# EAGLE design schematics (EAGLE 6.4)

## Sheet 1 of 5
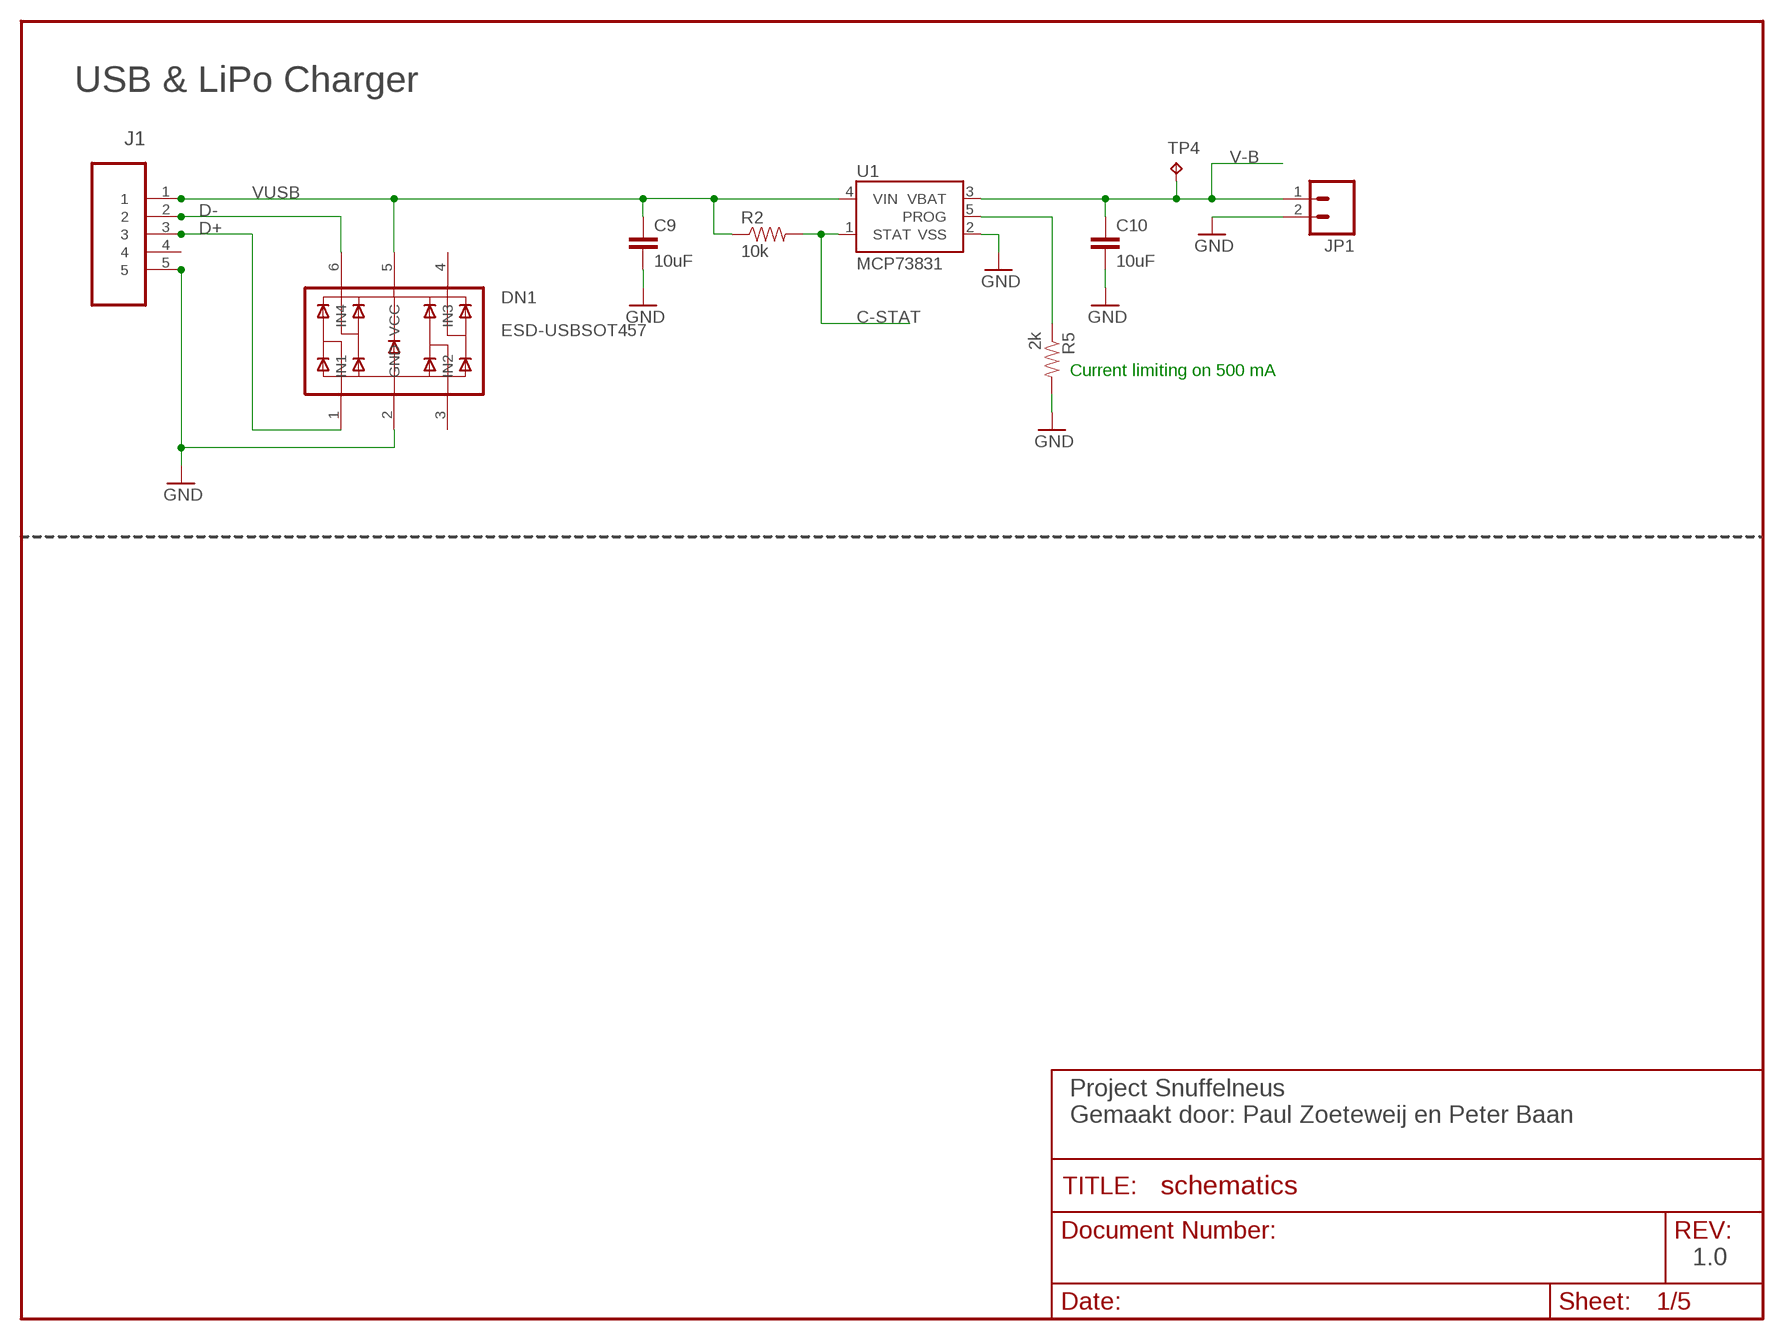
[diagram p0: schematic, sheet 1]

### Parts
C9  10uF  CAP0805  [0805]
C10  10uF  CAP0805  [0805]
DN1  ESD-USBSOT457  [SOT457]
J1  47346-0001  [MOLEX_47346-0001]
JP1  M02-JST-2MM-SMT  [S2B-PH]
R2  10k  RESISTOR  [0805]
R5  2k  RESISTOR  [0805]
TP4  TPTP20R  [TP20R]
U1  MCP73831  [SOT23-5]

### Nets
C-STAT: R2.2 U1.1(STAT) ; also sheet 3
D+: DN1.1(IN1) J1.3 ; also sheet 3
D-: DN1.6(IN4) J1.2 ; also sheet 3
GND: C9.2 C10.2 DN1.2(GND) J1.5 JP1.2 R5.2 U1.2(VSS) ; also sheet 2,3,4,5
N$11: R5.1 U1.5(PROG)
V-B: C10.1 JP1.1 TP4.TP U1.3(VBAT) ; also sheet 2
VUSB: C9.1 DN1.5(VCC) J1.1 R2.1 U1.4(VIN) ; also sheet 2
Unconnected: DN1.3(IN2) DN1.4(IN3) J1.4

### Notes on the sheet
- USB & LiPo Charger
- Current limiting on 500 mA
- Project Snuffelneus
  Gemaakt door: Paul Zoeteweij en Peter Baan
- 1.0

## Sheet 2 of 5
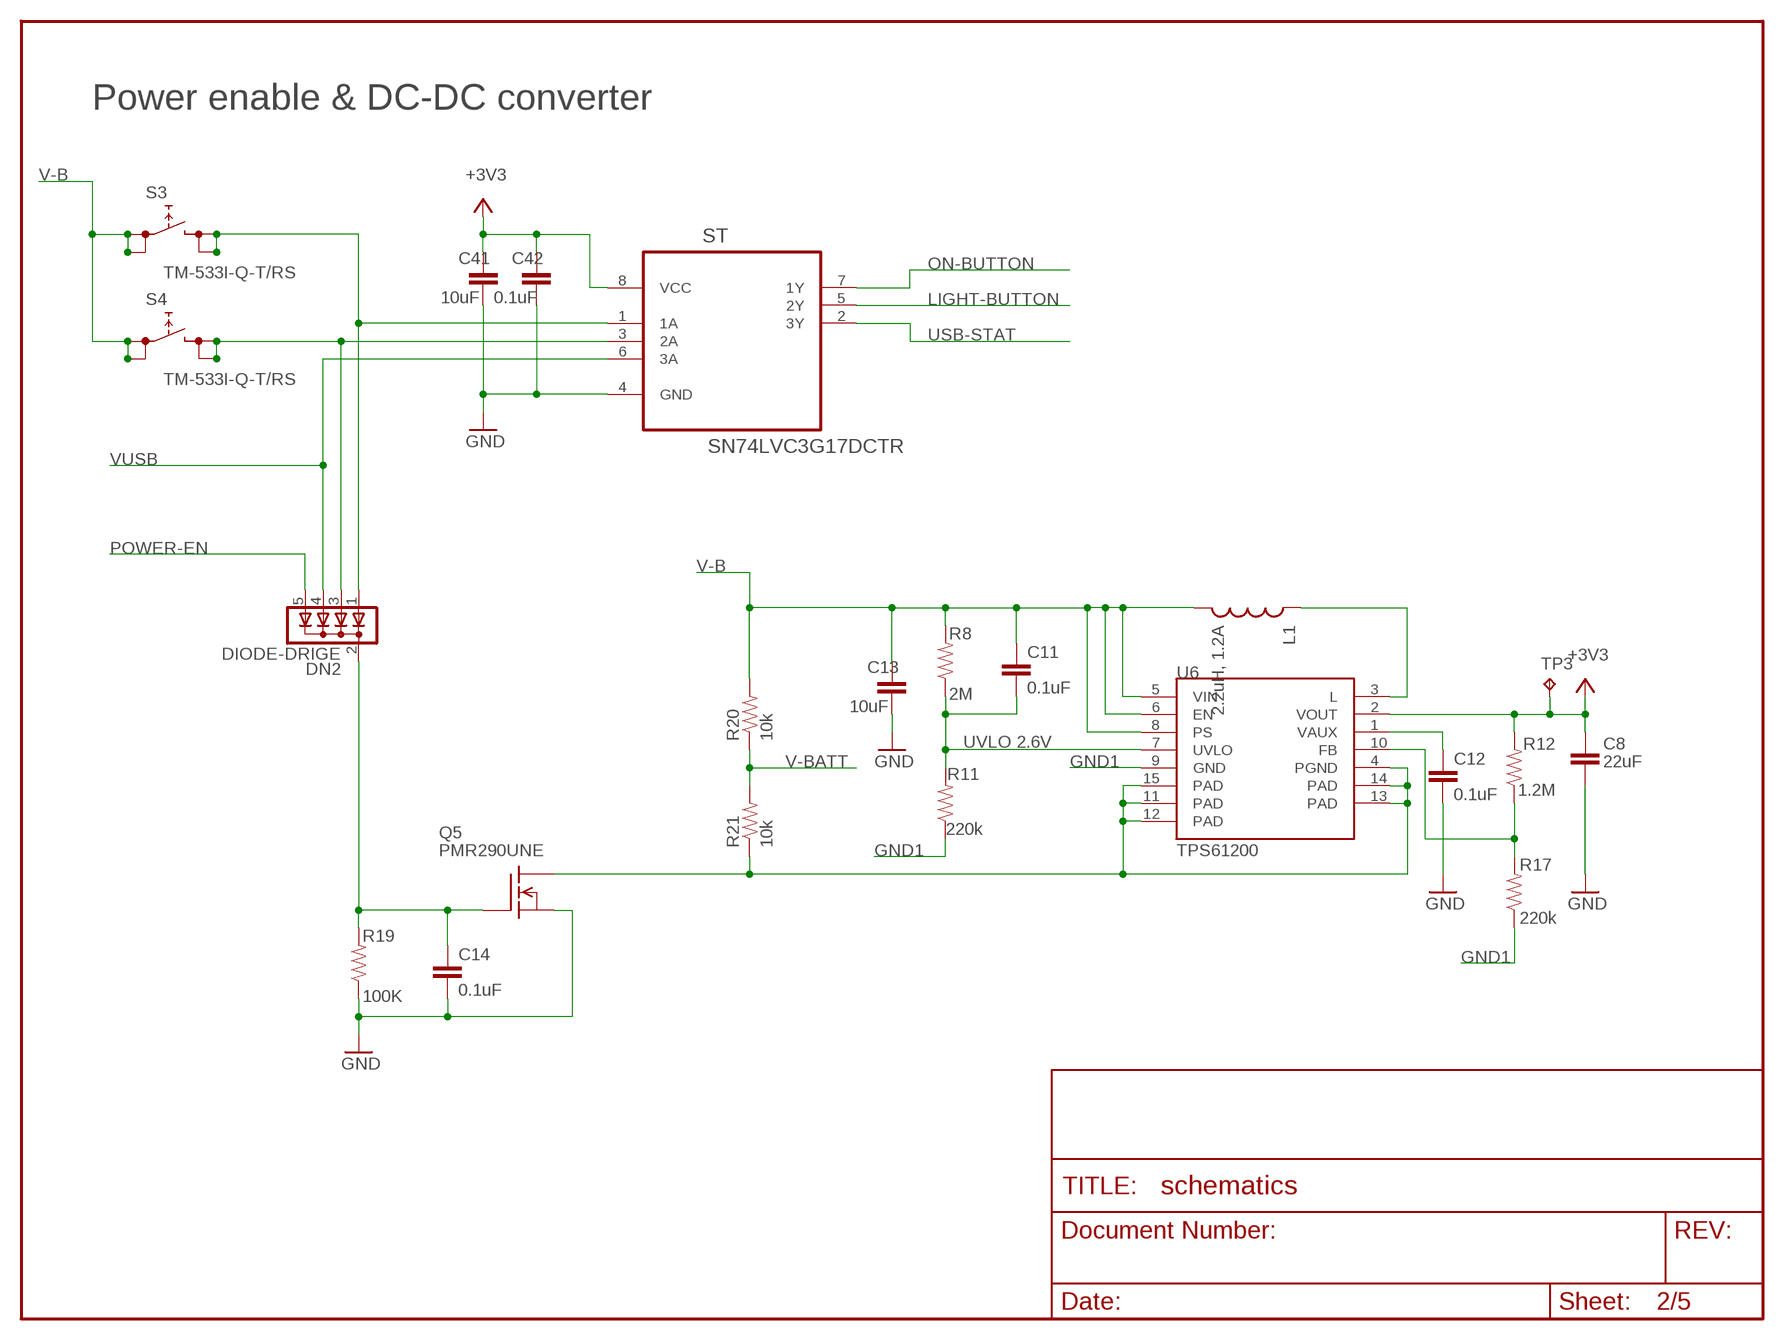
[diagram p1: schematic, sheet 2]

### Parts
C8  22uF  CAP0805  [0805]
C11  0.1uF  CAP0805  [0805]
C12  0.1uF  CAP0805  [0805]
C13  10uF  CAP0805  [0805]
C14  0.1uF  CAP0805  [0805]
C41  10uF  CAP0805  [0805]
C42  0.1uF  CAP0805  [0805]
DN2  DIODE-DRIGE  [SOT353]
L1  2.2uH, 1.2A  INDUCTORCR75  [LPS3015-222MLC]
Q5  PMR290UNE  [SOT23]
R8  2M  RESISTOR  [0805]
R11  220k  RESISTOR  [0805]
R12  1.2M  RESISTOR  [0805]
R17  220k  RESISTOR  [0805]
R19  100K  RESISTOR  [0805]
R20  10k  RESISTOR  [0805]
R21  10k  RESISTOR  [0805]
S3  TM-533I-Q-T/RS  [TM-533I-Q-T/R]
S4  TM-533I-Q-T/RS  [TM-533I-Q-T/R]
ST  SN74LVC3G17DCTR  [SOP65P400X130-8N]
TP3  TPTP20R  [TP20R]
U6  TPS61200  [QFN-10_PAD]

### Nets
3.3V1: R12.1 R17.2 U6.10(FB)
+3V3: C8.1 C41.1 C42.1 R12.2 ST.8(VCC) TP3.TP U6.2(VOUT) ; also sheet 3,4,5
GND: C8.2 C12.2 C13.2 C14.2 C41.2 C42.2 Q5.2(S) R19.1 ST.4(GND) ; also sheet 1,3,4,5
GND1: R11.1 R17.1 U6.9(GND)
LIGHT-BUTTON: ST.5(2Y) ; also sheet 3
LIGHT/WAKEUP-BUTTON1: DN2.3(A2) S4.T3 S4.T4 ST.3(2A)
N$8: L1.P$1 U6.3(L)
N$9: C12.1 U6.1(VAUX)
N$10: C14.1 DN2.2(C) Q5.1(G) R19.2
ON-BUTTON: ST.7(1Y) ; also sheet 3
PAD@4: Q5.3(D) R21.1 U6.4(PGND) U6.11(PAD) U6.12(PAD) U6.13(PAD) U6.14(PAD) U6.15(PAD)
POWER-EN: DN2.5(A4) ; also sheet 3
USB-STAT: ST.2(3Y) ; also sheet 3
UVLO1: C11.2 R8.1 R11.2 U6.7(UVLO)
V-B: C11.1 C13.1 L1.P$2 R8.2 R20.2 S3.T1 S3.T2 S4.T1 S4.T2 U6.5(VIN) U6.6(EN) U6.8(PS) ; also sheet 1
V-BATT: R20.1 R21.2 ; also sheet 3
VUSB: DN2.4(A3) ST.6(3A) ; also sheet 1
WAKEUP-BUTTON1: DN2.1(A1) S3.T3 S3.T4 ST.1(1A)

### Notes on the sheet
- Power enable & DC-DC converter
- UVLO 2.6V

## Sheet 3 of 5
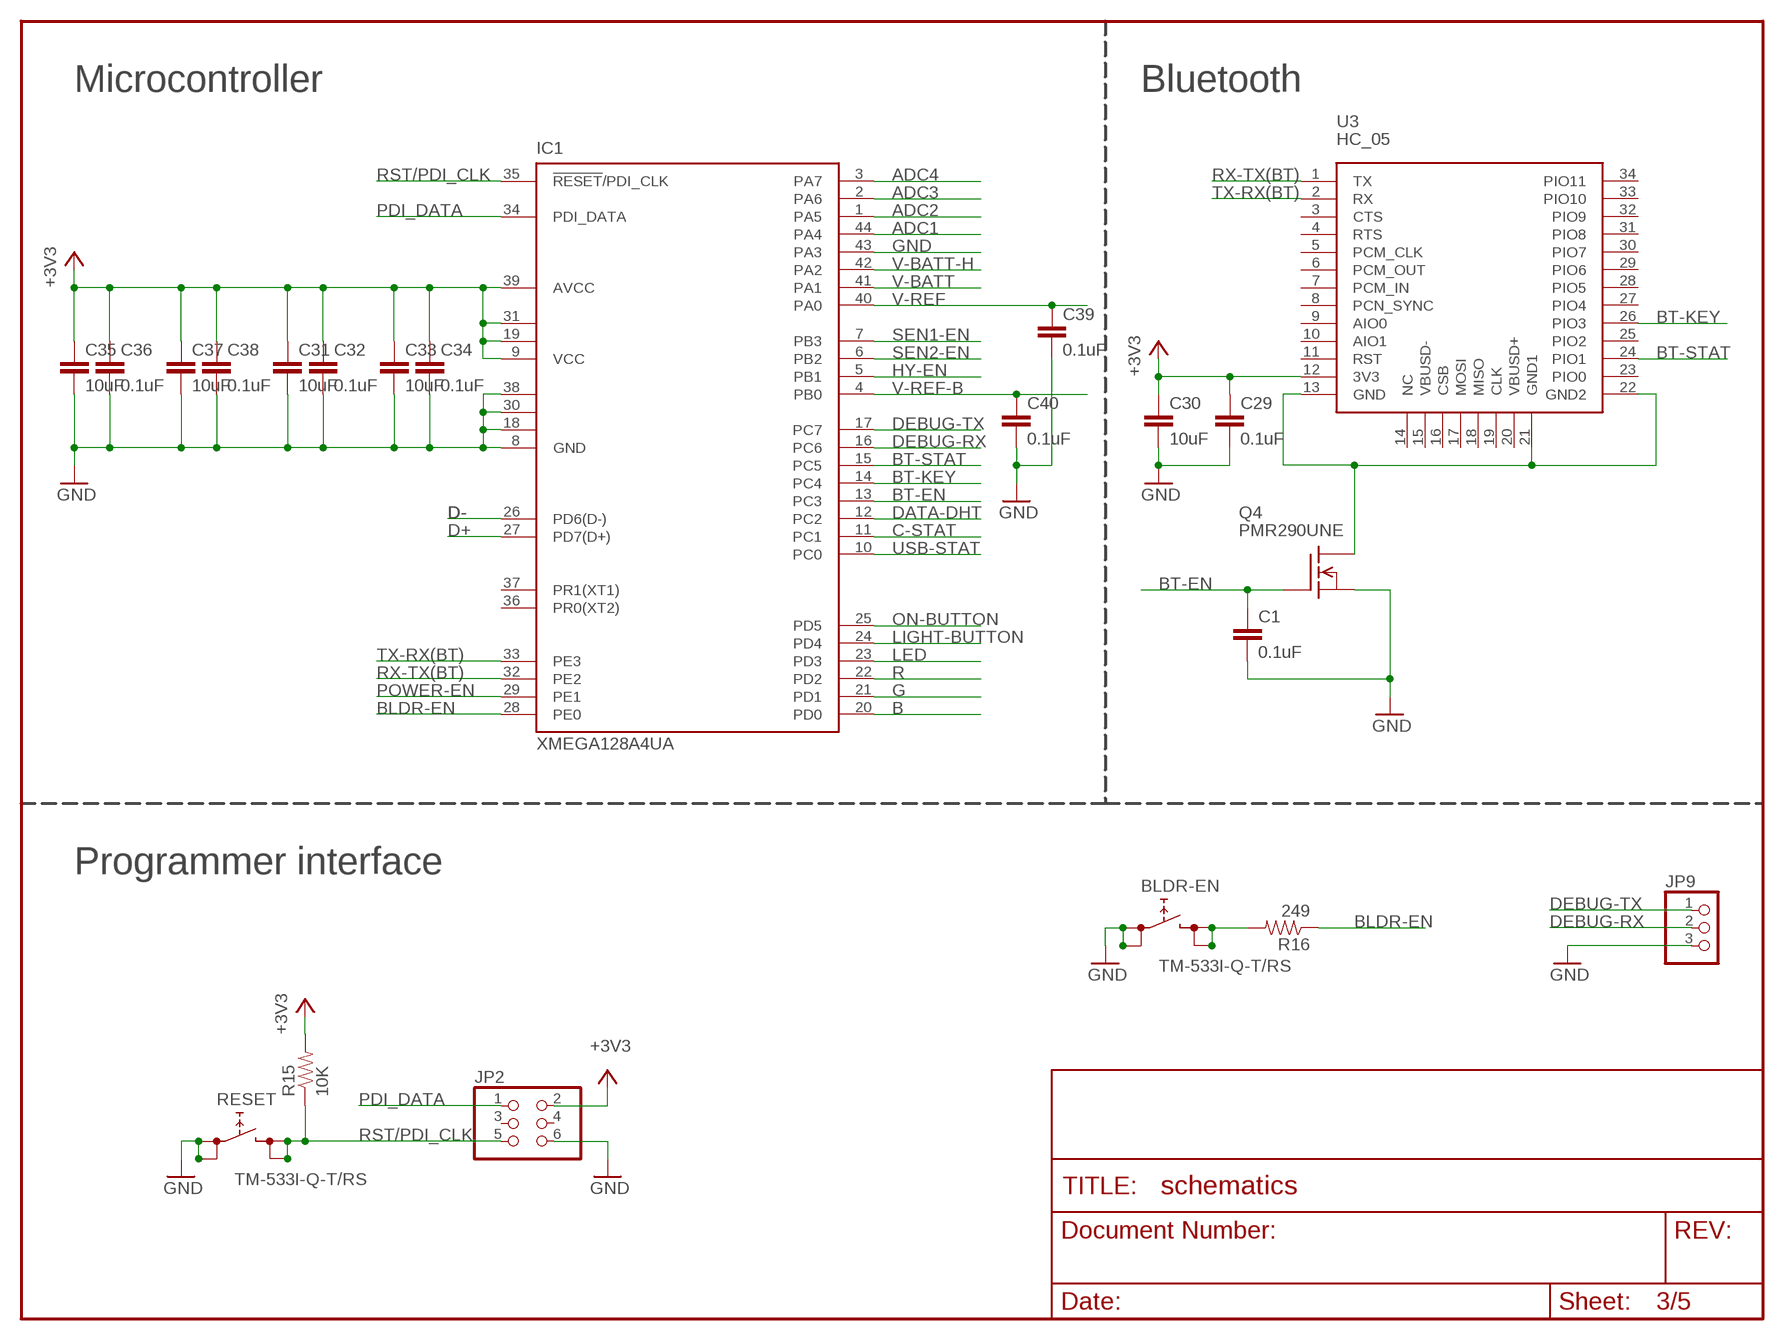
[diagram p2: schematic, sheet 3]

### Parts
BLDR-EN  TM-533I-Q-T/RS  [TM-533I-Q-T/R]
C1  0.1uF  CAP0805  [0805]
C29  0.1uF  CAP0805  [0805]
C30  10uF  CAP0805  [0805]
C31  10uF  CAP0805  [0805]
C32  0.1uF  CAP0805  [0805]
C33  10uF  CAP0805  [0805]
C34  0.1uF  CAP0805  [0805]
C35  10uF  CAP0805  [0805]
C36  0.1uF  CAP0805  [0805]
C37  10uF  CAP0805  [0805]
C38  0.1uF  CAP0805  [0805]
C39  0.1uF  CAP0805  [0805]
C40  0.1uF  CAP0805  [0805]
IC1  XMEGA128A4UA  [TQFP44]
JP2  PINHD-2X3  [2X03]
JP9  PINHD-1X3  [1X03]
Q4  PMR290UNE  [SOT23]
R15  10K  RESISTOR  [0805]
R16  249  RESISTOR  [0805]
RESET  TM-533I-Q-T/RS  [TM-533I-Q-T/R]
U3  HC_05  [BLUETOOTH_SMD]

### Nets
+3V3: C29.1 C30.1 C31.1 C32.1 C33.1 C34.1 C35.1 C36.1 C37.1 C38.1 IC1.9(VCC) IC1.19(VCC1) IC1.31(VCC2) IC1.39(AVCC) JP2.2 R15.2 U3.12(3V3) ; also sheet 2,4,5
ADC1: IC1.44(PA4) ; also sheet 4
ADC2: IC1.1(PA5) ; also sheet 4
ADC3: IC1.2(PA6) ; also sheet 4
ADC4: IC1.3(PA7) ; also sheet 4
B: IC1.20(PD0) ; also sheet 5
BLDR-EN: IC1.28(PE0) R16.1
BT-EN: C1.1 IC1.13(PC3) Q4.1(G)
BT-KEY: IC1.14(PC4) U3.26(PIO3)
BT-STAT: IC1.15(PC5) U3.24(PIO1)
C-STAT: IC1.11(PC1) ; also sheet 1
D+: IC1.27(PD7(D+)) ; also sheet 1
D-: IC1.26(PD6(D-)) ; also sheet 1
DATA-DHT: IC1.12(PC2) ; also sheet 5
DEBUG-RX: IC1.16(PC6) JP9.2
DEBUG-TX: IC1.17(PC7) JP9.1
G: IC1.21(PD1) ; also sheet 5
GND: BLDR-EN.T1 BLDR-EN.T2 C1.2 C29.2 C30.2 C31.2 C32.2 C33.2 C34.2 C35.2 C36.2 C37.2 C38.2 C39.2 C40.2 IC1.8(GND) IC1.18(GND1) IC1.30(GND2) IC1.38(GND3) IC1.43(PA3) JP2.6 JP9.3 Q4.2(S) RESET.T1 RESET.T2 ; also sheet 1,2,4,5
HY-EN: IC1.5(PB1) ; also sheet 4
LED: IC1.23(PD3) ; also sheet 5
LIGHT-BUTTON: IC1.24(PD4) ; also sheet 2
N$4: Q4.3(D) U3.13(GND) U3.21(GND1) U3.22(GND2)
N$5: BLDR-EN.T3 BLDR-EN.T4 R16.2
ON-BUTTON: IC1.25(PD5) ; also sheet 2
PDI_DATA: IC1.34(PDI_DATA) JP2.1
POWER-EN: IC1.29(PE1) ; also sheet 2
R: IC1.22(PD2) ; also sheet 5
RST/PDI_CLK: IC1.35(!RESET!/PDI_CLK) JP2.5 R15.1 RESET.T3 RESET.T4
RX-TX(BT): IC1.32(PE2) U3.1(TX)
SEN1-EN: IC1.7(PB3) ; also sheet 5
SEN2-EN: IC1.6(PB2) ; also sheet 4
TX-RX(BT): IC1.33(PE3) U3.2(RX)
USB-STAT: IC1.10(PC0) ; also sheet 2
V-BATT: IC1.41(PA1) ; also sheet 2
V-BATT-H: IC1.42(PA2) ; also sheet 4
V-REF: C39.1 IC1.40(PA0) ; also sheet 4
V-REF-B: C40.1 IC1.4(PB0) ; also sheet 4
Unconnected: IC1.36(PR0(XT2)) IC1.37(PR1(XT1)) JP2.3 JP2.4 U3.3(CTS) U3.4(RTS) U3.5(PCM_CLK) U3.6(PCM_OUT) U3.7(PCM_IN) U3.8(PCN_SYNC) U3.9(AIO0) U3.10(AIO1) U3.11(RST) U3.14(NC) U3.15(VBUSD-) U3.16(CSB) U3.17(MOSI) U3.18(MISO) U3.19(CLK) U3.20(VBUSD+) U3.23(PIO0) U3.25(PIO2) U3.27(PIO4) U3.28(PIO5) U3.29(PIO6) U3.30(PIO7) U3.31(PIO8) U3.32(PIO9) U3.33(PIO10) U3.34(PIO11)

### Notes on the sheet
- Microcontroller | Bluetooth
- Programmer interface

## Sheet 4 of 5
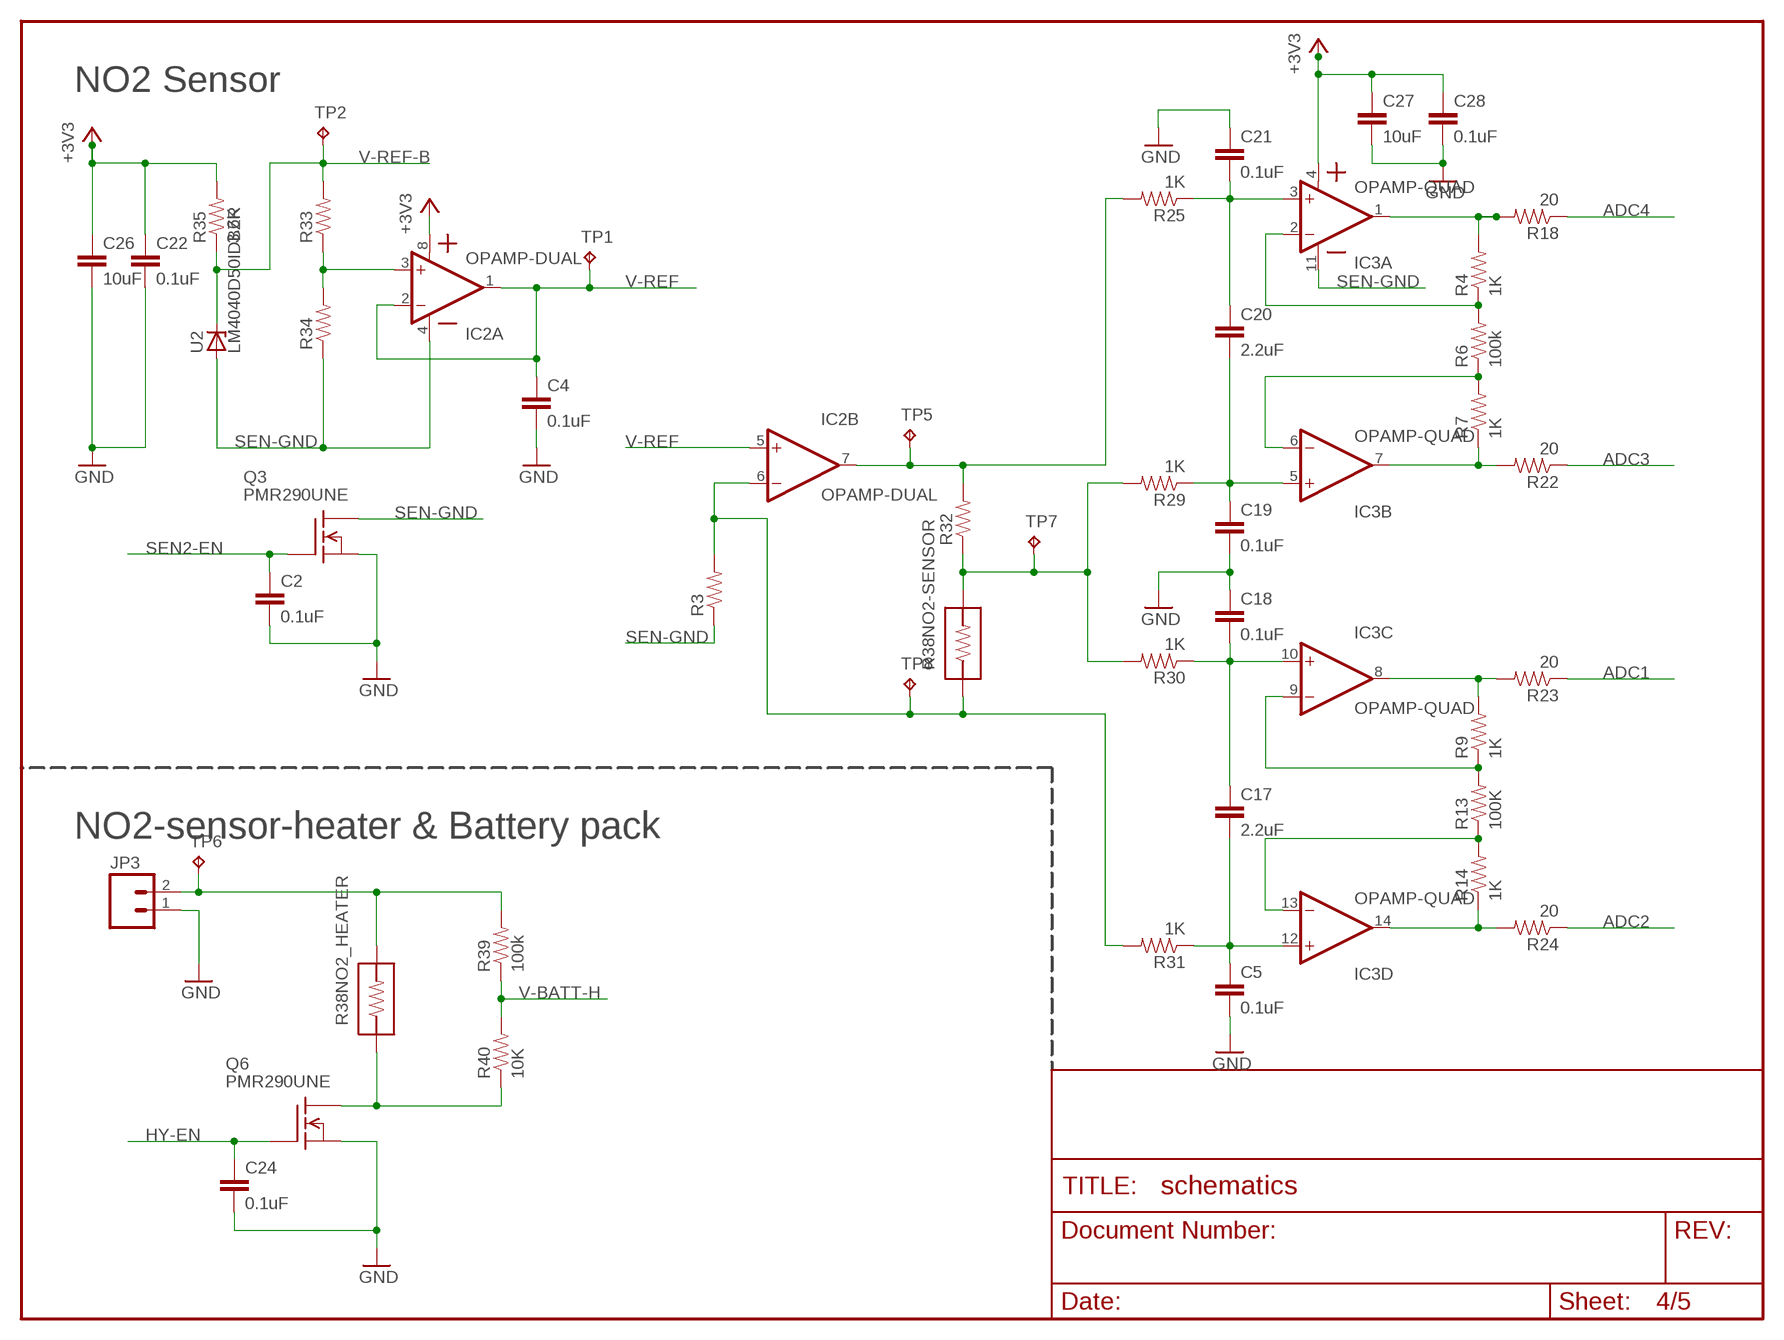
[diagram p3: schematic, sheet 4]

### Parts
C2  0.1uF  CAP0805  [0805]
C4  0.1uF  CAP0805  [0805]
C5  0.1uF  CAP0805  [0805]
C17  2.2uF  CAP0805  [0805]
C18  0.1uF  CAP0805  [0805]
C19  0.1uF  CAP0805  [0805]
C20  2.2uF  CAP0805  [0805]
C21  0.1uF  CAP0805  [0805]
C22  0.1uF  CAP0805  [0805]
C24  0.1uF  CAP0805  [0805]
C26  10uF  CAP0805  [0805]
C27  10uF  CAP0805  [0805]
C28  0.1uF  CAP0805  [0805]
IC2  OPAMP-DUAL  [SOIC127P600X175-8N]
IC3  OPAMP-QUAD  [SOIC127P600X175-14N]
JP3  M025MM  [SCREWTERMINAL-5MM-2]
Q3  PMR290UNE  [SOT23]
Q6  PMR290UNE  [SOT23]
R3  RESISTOR  [0805]
R4  1K  RESISTOR  [0805]
R6  100k  RESISTOR  [0805]
R7  1K  RESISTOR  [0805]
R9  1K  RESISTOR  [0805]
R13  100K  RESISTOR  [0805]
R14  1K  RESISTOR  [0805]
R18  20  RESISTOR  [0805]
R22  20  RESISTOR  [0805]
R23  20  RESISTOR  [0805]
R24  20  RESISTOR  [0805]
R25  1K  RESISTOR  [0805]
R29  1K  RESISTOR  [0805]
R30  1K  RESISTOR  [0805]
R31  1K  RESISTOR  [0805]
R32  RESISTOR  [0805]
R33  RESISTOR  [0805]
R34  RESISTOR  [0805]
R35  3.6K  RESISTOR  [0805]
R38  NO2-SENSOR  [DIP08]
R39  100k  RESISTOR  [0805]
R40  10K  RESISTOR  [0805]
TP1  TPTP20R  [TP20R]
TP2  TPTP20R  [TP20R]
TP5  TPTP20R  [TP20R]
TP6  TPTP20R  [TP20R]
TP7  TPTP20R  [TP20R]
TP8  TPTP20R  [TP20R]
U2  LM4040D50IDBZR  [SOT95P237X112-3N]

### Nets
+3V3: C22.1 C26.1 C27.1 C28.1 IC2.8(A:VDD) IC3.4(A:VDD) R35.2 ; also sheet 2,3,5
ADC1: R23.1 ; also sheet 3
ADC2: R24.1 ; also sheet 3
ADC3: R22.1 ; also sheet 3
ADC4: R18.1 ; also sheet 3
GND: C2.2 C4.2 C5.2 C18.1 C19.2 C21.1 C22.2 C24.2 C26.2 C27.2 C28.2 JP3.1 Q3.2(S) Q6.2(S) ; also sheet 1,2,3,5
HY-EN: C24.1 Q6.1(G) ; also sheet 3
N$1: IC3.2(A:-IN) R4.1 R6.2
N$2: IC3.6(B:-IN) R6.1 R7.2
N$7: IC3.9(C:-IN) R9.1 R13.2
N$12: IC3.13(D:-IN) R13.1 R14.2
N$14: IC3.1(A:OUT) R4.2 R18.2
N$15: IC3.7(B:OUT) R7.1 R22.2
N$19: IC3.8(C:OUT) R9.2 R23.2
N$21: IC3.14(D:OUT) R14.1 R24.2
N$22: C17.1 C18.2 IC3.10(C:+IN) R30.1
N$23: IC2.3(A:+IN) R33.1 R34.2
N$25: C19.1 C20.2 IC3.5(B:+IN) R29.1
N$26: C20.1 C21.2 IC3.3(A:+IN) R25.1
N$27: C5.1 C17.2 IC3.12(D:+IN) R31.1
N$28: JP3.2 R38.8 R39.2 TP6.TP
N$29: Q6.3(D) R38.1 R40.1
N$33: R29.2 R30.2 R32.1 R38.7 TP7.TP
N$34: IC2.7(B:OUT) R25.2 R32.2 TP5.TP
N$35: IC2.6(B:-IN) R3.2 R31.2 R38.2 TP8.TP
SEN2-EN: C2.1 Q3.1(G) ; also sheet 3
SEN-GND: IC2.4(A:GND) IC3.11(A:GND) Q3.3(D) R3.1 R34.1 U2.2(A)
V-BATT-H: R39.1 R40.2 ; also sheet 3
V-REF: C4.1 IC2.1(A:OUT) IC2.2(A:-IN) IC2.5(B:+IN) TP1.TP ; also sheet 3
V-REF-B: R33.2 R35.1 TP2.TP U2.1(C) ; also sheet 3

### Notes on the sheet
- NO2 Sensor
- NO2-sensor-heater & Battery pack

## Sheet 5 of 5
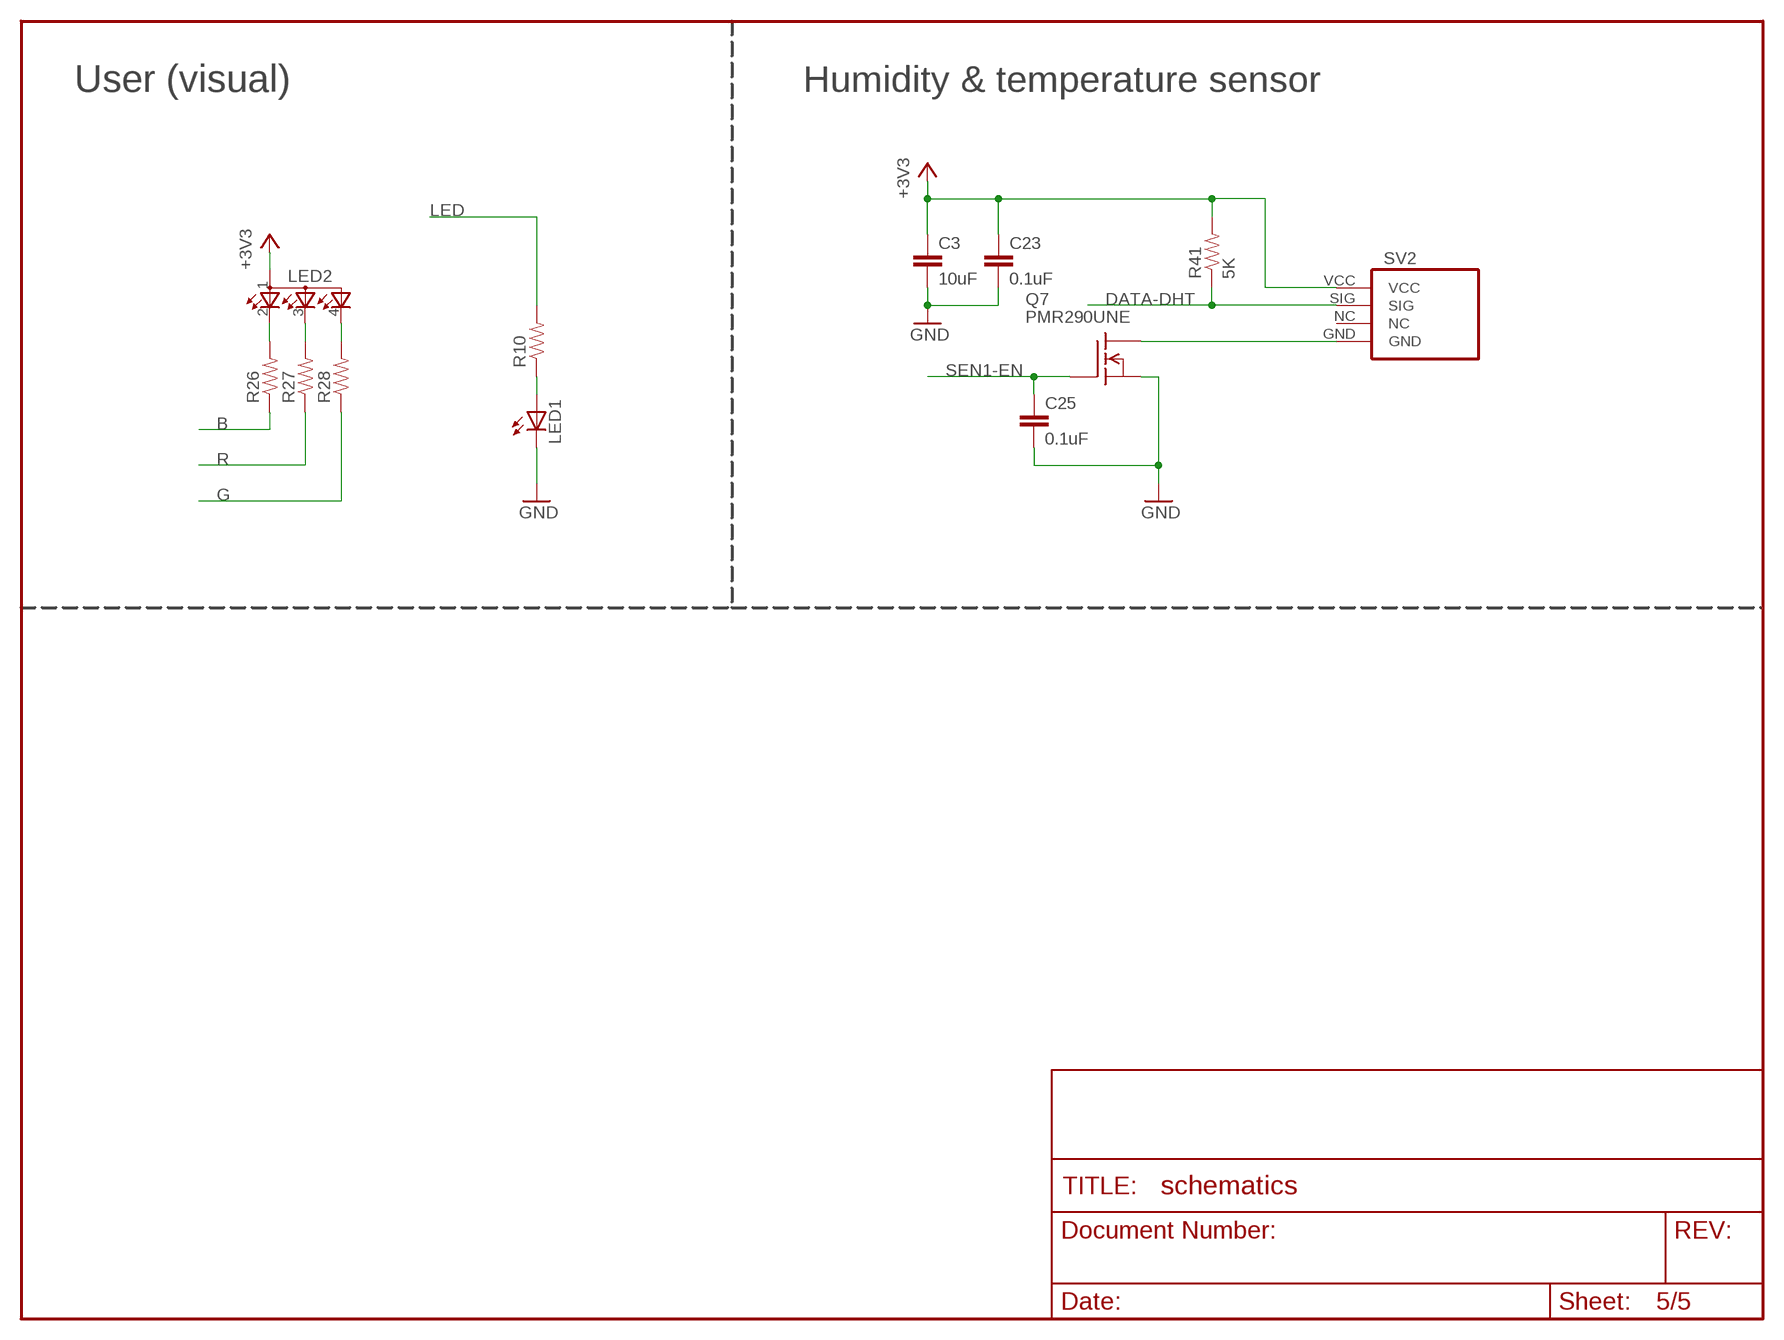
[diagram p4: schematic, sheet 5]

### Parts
C3  10uF  CAP0805  [0805]
C23  0.1uF  CAP0805  [0805]
C25  0.1uF  CAP0805  [0805]
LED1  LED5MM  [LED5MM]
LED2  RGBLED  [150141M173100]
Q7  PMR290UNE  [SOT23]
R10  RESISTOR  [0805]
R26  RESISTOR  [0805]
R27  RESISTOR  [0805]
R28  RESISTOR  [0805]
R41  5K  RESISTOR  [0805]
SV2  DHT11  [DHT11]

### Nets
435: LED2.3(3R) R27.2
+3V3: C3.1 C23.1 LED2.1 R41.2 SV2.VCC ; also sheet 2,3,4
B: R26.1 ; also sheet 3
B2: LED2.2(2B) R26.2
DATA-DHT: R41.1 SV2.SIG ; also sheet 3
G: R28.1 ; also sheet 3
G2: LED2.4(4G) R28.2
GND: C3.2 C23.2 C25.2 LED1.K(C) Q7.2(S) ; also sheet 1,2,3,4
LED: R10.2 ; also sheet 3
N$6: LED1.A R10.1
N$30: Q7.3(D) SV2.GND
R: R27.1 ; also sheet 3
SEN1-EN: C25.1 Q7.1(G) ; also sheet 3
Unconnected: SV2.NC

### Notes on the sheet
- User (visual) | Humidity & temperature sensor

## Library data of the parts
BLDR-EN RESET S3 S4 = snuffelneus:TM-533I-Q-T/R: 6.2 X 6.5mm TACT Switch (SMD) Source: http://www3.alps.co.jp/WebObjects/catalog.woa/PDF/E/Switch/Tact/SKHM/SKHM.PDF
C1-C5 C9-C12 C14 C17-C40 = SparkFun:CAP: Capacitor
C8 C13 C41 C42 = CH_passive:CAP: Capacitor
DN1 = snuffelneus:ESD-USB: 4 DIODES SIL, common cathode
DN2 = snuffelneus:DIODE-DRIGE: 4 DIODES SIL, common cathode
IC1 = snuffelneus:XMEGA128A4U: MICROCONTROLLER Features High-performance, Low-power 8/16-bit AVR XMEGA Microcontroller Non-Volatile Program and Data Memories - 16 KB - 128 KB of In-System Self-Programmable Flash - 4 KB - 8 KB Boot Code Section with Independent Lock Bits - 1 KB - 2 KB EEPROM - 2 KB - 8 KB Internal SRAM Peripheral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; OC_FARNELL: unknown; OC_NEWARK: unknown
IC2 = snuffelneus:OPAMP-DUAL: Operational Amplifier
IC3 = snuffelneus:OPAMP-QUAD: Operational Amplifier
J1 = Molex-47346-0001:47346-0001: CONN RCPT 5POS MICRO USB R/A SMD; MPN: 47346-0001; OC_FARNELL: 1568026; OC_NEWARK: 47M0505; PACKAGE: 5 POS MICRO USB R/A; SUPPLIER: MOLEX
JP1 JP3 = SparkFun:M02: Header 2
JP2 = pinhead:PINHD-2X3: PIN HEADER
JP9 = pinhead:PINHD-1X3: PIN HEADER
L1 = snuffelneus:INDUCTOR: Inductors
LED1 = led:LED: LED
LED2 = snuffelneus:RGBLED: OSRAM - Hyper Multi TOPLED® (RGB) LB E673, LV E673, LT E673 - Power TOPLED® Enhanced optical Power LED (HOP2000) LS E67B, LA E67B, LO E67B, LY E67B - Hyper Multi TOPLED® Enhanced optical Power LED (HOP2000 / ATON®) LATB T66B - Hyper Multi TOPLED® Hyper-Bright LED LATB T686 Source: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
Q3-Q7 = snuffelneus:PMR290UNE: N-Channel Enhancement MOSFET 200V; 1.5A; 1,6Ohm
R2-R35 R39-R41 = SparkFun:RESISTOR: Resistor
R38 = snuffelneus:NO2-SENSOR: Resistor Basic schematic elements and footprints for 0603, 1206, and PTH 1/10th watt (small) resistors.
ST = snuffelneus:SN74LVC3G17DCTR: TRIPLE SCHMITT-TRIGGER BUFFER; MPN: SN74LVC3G17DCTR; OC_FARNELL: 1236391; OC_NEWARK: 90H3713; PACKAGE: SSOP-8; SUPPLIER: Texas Instruments
SV2 = snuffelneus:DHT11: PIN HEADER
TP1-TP8 = testpad:TP: Test pad
U1 = SparkFun:MCP73831: Microchip's MCP73831 Miniature single cell, fully integrated Li-Ion, Li-polymer charge management controller http://ww1.microchip.com/downloads/en/DeviceDoc/21984a.pdf
U2 = snuffelneus:LM4040D50IDBZR: PRECISION MICROPOWER SHUNT VOLTAGE REFERENCE; MPN: LM4040D50IDBZR; OC_FARNELL: 1652239; OC_NEWARK: 43K3367; PACKAGE: 3-SOT-23; SUPPLIER: TEXAS INSTRUMENTS
U3 = SerialPortBluetooth:HC_05
U6 = SparkFun:TPS61200: DC to DC Booster

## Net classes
0 default: clearance 0.15 mm

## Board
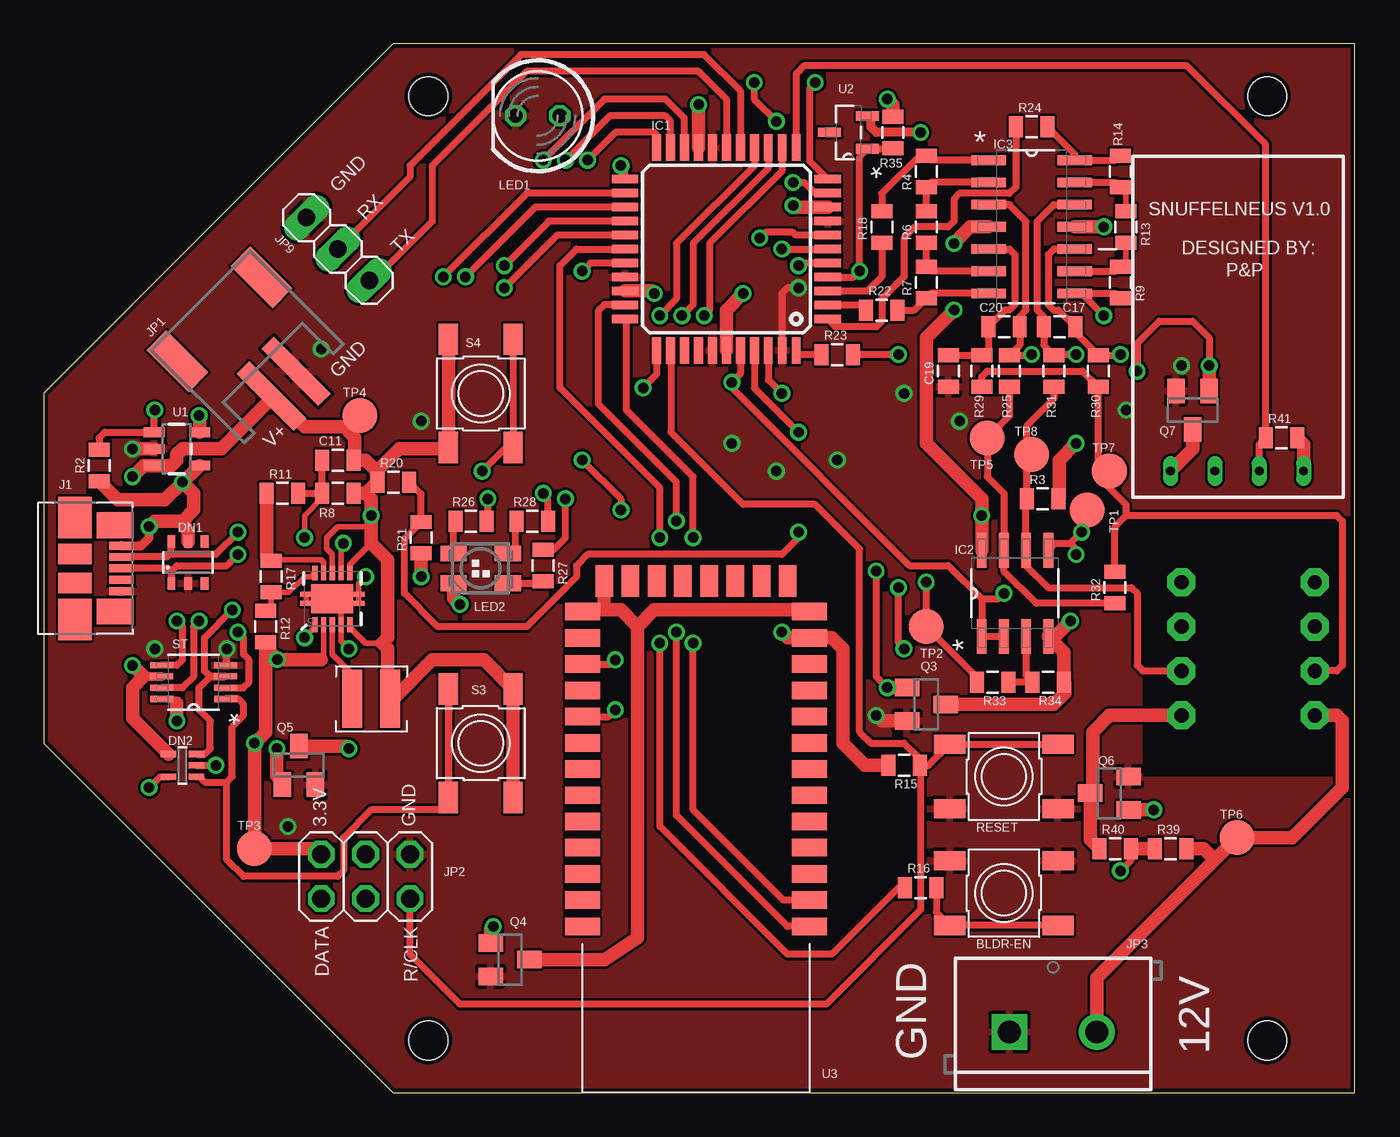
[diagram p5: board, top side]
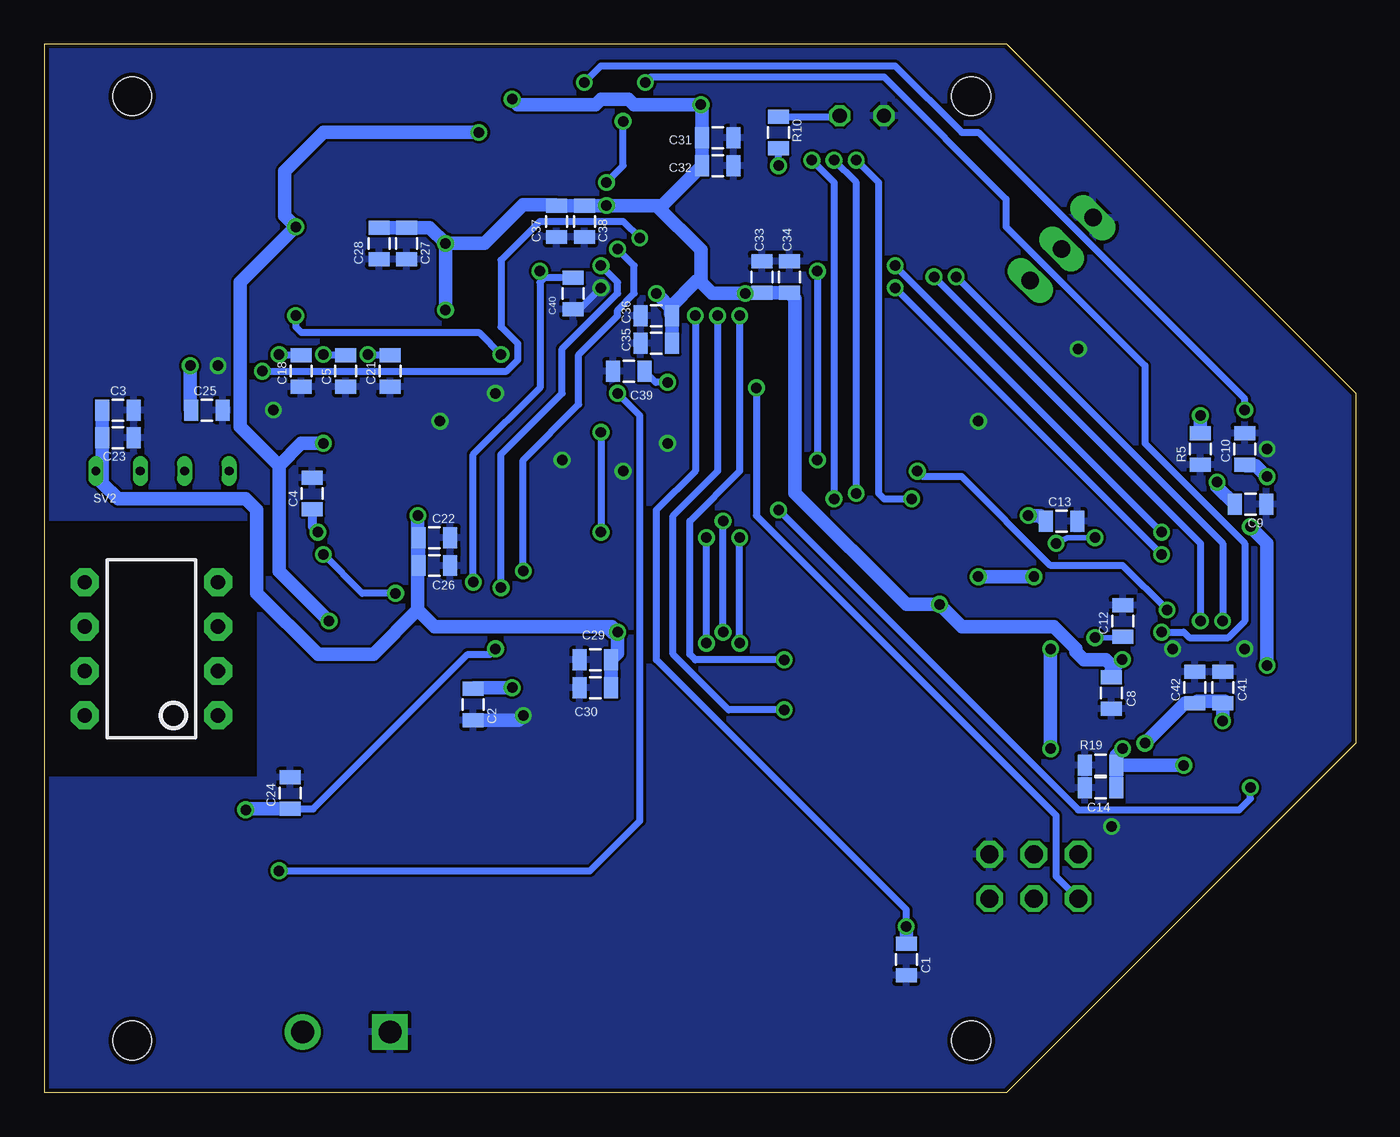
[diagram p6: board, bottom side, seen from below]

Size 75 x 60 mm. Coordinates in mm from the lower left corner, seen from the top.
Outline: 0,20 20,0 75,0 75,60 20,60 0,40 0,20
Copper layers (1*16): Top 0.018mm / dielectric 1.55mm / Bottom 0.018mm
Design rules "eC_2Layer_PClass6_BaseCopperO18_eCDefault *": minimum track width 0.15mm, minimum drill 0.35mm, track to track 0.15mm, track to pad 0.15mm, pad to pad 0.15mm, via to via 0.15mm, smd to smd 0mil, copper to edge 0.25mm, drill to drill 0.35mm, minimum pad ring 0.175mm, minimum via ring 0.125mm, stop-mask expansion 0mil, vias tented up to drill 0.45mm, thermal gap 0.2mm
Holes 2.2 mm at 70,57 22,57 22,3 70,3
tRestrict: area 62.9,18.1 to 74.9,32.7
bRestrict: area 62.9,18.1 to 74.9,32.7

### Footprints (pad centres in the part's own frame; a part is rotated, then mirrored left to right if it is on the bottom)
TM-533I-Q-T/R = smd 1.8 x 1.1: T1 -3.1,1.85; T2 3.1,1.85; T3 -3.1,-1.85; T4 3.1,-1.85
0805 = smd 0.8 x 1.2: 1 -0.9,0; 2 0.9,0
SOT457 = smd 0.7 x 0.45: 1 -1.2,0.95; 2 -1.2,0; 3 -1.2,-0.95; 4 1.2,-0.95; 5 1.2,0; 6 1.2,0.95
SOT353 = smd 0.35 x 0.9: 1 -0.65,-0.8; 2 0,-0.8; 3 0.65,-0.8; 4 0.65,0.8; 5 -0.65,0.8
TQFP44 = smd 1.5 x 0.5: 1 -5.8,4; 2 -5.8,3.2; 3 -5.8,2.4; 4 -5.8,1.6; 5 -5.8,0.8; 6 -5.8,0; 7 -5.8,-0.8; 8 -5.8,-1.6; 9 -5.8,-2.4; 10 -5.8,-3.2; 11 -5.8,-4; 23 5.8,-4; 24 5.8,-3.2; 25 5.8,-2.4; 26 5.8,-1.6; 27 5.8,-0.8; 28 5.8,0; 29 5.8,0.8; 30 5.8,1.6; 31 5.8,2.4; 32 5.8,3.2; 33 5.8,4 | smd 0.5 x 1.5: 12 -4,-5.8; 13 -3.2,-5.8; 14 -2.4,-5.8; 15 -1.6,-5.8; 16 -0.8,-5.8; 17 0,-5.8; 18 0.8,-5.8; 19 1.6,-5.8; 20 2.4,-5.8; 21 3.2,-5.8; 22 4,-5.8; 34 4,5.8; 35 3.2,5.8; 36 2.4,5.8; 37 1.6,5.8; 38 0.8,5.8; 39 0,5.8; 40 -0.8,5.8; 41 -1.6,5.8; 42 -2.4,5.8; 43 -3.2,5.8; 44 -4,5.8
SOIC127P600X175-8N = smd 1.981 x 0.559: 1 -2.464,1.905; 2 -2.464,0.635; 3 -2.464,-0.635; 4 -2.464,-1.905; 5 2.464,-1.905; 6 2.464,-0.635; 7 2.464,0.635; 8 2.464,1.905
SOIC127P600X175-14N = smd 1.981 x 0.559: 1 -2.464,3.81; 2 -2.464,2.54; 3 -2.464,1.27; 4 -2.464,0; 5 -2.464,-1.27; 6 -2.464,-2.54; 7 -2.464,-3.81; 8 2.464,-3.81; 9 2.464,-2.54; 10 2.464,-1.27; 11 2.464,0; 12 2.464,1.27; 13 2.464,2.54; 14 2.464,3.81
MOLEX_47346-0001 = smd 0.45 x 1.38: 1 -1.3,0; 2 -0.65,0; 3 0,0; 4 0.65,0; 5 1.3,0 | smd 1.475 x 2.1: M1 -2.462,-0.36; M2 2.462,-0.36 | smd 2.375 x 1.9: M3 -2.913,-2.66; M6 2.913,-2.66 | smd 1.175 x 1.9: M4 -0.82,-2.66; M5 0.85,-2.66
S2B-PH = smd 1 x 4.6: 1 -1,-3.7; 2 1,-3.7 | smd 1.6 x 3.4: NC1 -3.4,1.5; NC2 3.4,1.5
2X03 = drill 1.016 octagon: 1 -2.54,-1.27; 2 -2.54,1.27; 3 0,-1.27; 4 0,1.27; 5 2.54,-1.27; 6 2.54,1.27
SCREWTERMINAL-5MM-2 = drill 1.3 pad 2.032 square: 1 0,0 | drill 1.3 pad 2.032: 2 5,0
1X03 = drill 1.016 long: 1 -2.54,0; 2 0,0; 3 2.54,0
LPS3015-222MLC = smd 1.143 x 3.302: P$1 -1.079,0; P$2 1.079,0
LED5MM = drill 0.813 octagon: A -1.27,0; K 1.27,0
150141M173100 = smd 1.5 x 0.9: 1 1.55,0.85; 2 1.55,-0.85; 3 -1.55,0.85; 4 -1.55,-0.85
SOT23 = smd 1 x 1.4: 1 -0.95,-1.1; 2 0.95,-1.1; 3 0,1.1
DIP08 = drill 0.813 pad 1.6 octagon: 1 -3.81,-3.81; 2 -1.27,-3.81; 3 1.27,-3.81; 4 3.81,-3.81; 5 3.81,3.81; 6 1.27,3.81; 7 -1.27,3.81; 8 -3.81,3.81
SOP65P400X130-8N = smd 1.321 x 0.356: 1 -1.829,0.965; 2 -1.829,0.33; 3 -1.829,-0.33; 4 -1.829,-0.965; 5 1.829,-0.965; 6 1.829,-0.33; 7 1.829,0.33; 8 1.829,0.965
DHT11 = drill 0.5 pad 0.698 long: GND 0,-7.62; NC 0,-5.08; SIG 0,-2.54; VCC 0,0
TP20R = smd 2 x 2: TP 0,0
SOT23-5 = smd 0.55 x 1.2: 1 -0.95,-1.3; 2 0,-1.3; 3 0.95,-1.3; 4 0.95,1.3; 5 -0.95,1.3
SOT95P237X112-3N = smd 1.321 x 0.559: 1 -1.092,0.94; 2 -1.092,-0.94 | smd 1.321 x 0.508: 3 1.092,0
BLUETOOTH_SMD = smd 2 x 1: 1 0,0; 2 0,-1.5; 3 0,-3; 4 0,-4.5; 5 0,-6; 6 0,-7.5; 7 0,-9; 8 0,-10.5; 9 0,-12; 10 0,-13.5; 11 0,-15; 12 0,-16.5; 13 0,-18; 22 13,-18; 23 13,-16.5; 24 13,-15; 25 13,-13.5; 26 13,-12; 27 13,-10.5; 28 13,-9; 29 13,-7.5; 30 13,-6; 31 13,-4.5; 32 13,-3; 33 13,-1.5; 34 13,0 | smd 1 x 1.8: 14 1.25,-19.75; 15 2.75,-19.75; 16 4.25,-19.75; 17 5.75,-19.75; 18 7.25,-19.75; 19 8.75,-19.75; 20 10.25,-19.75; 21 11.75,-19.75
QFN-10_PAD = smd 0.297 x 0.85: 1 -1,-1.475; 2 -0.5,-1.475; 3 0,-1.475; 4 0.5,-1.475; 5 1,-1.475; 6 1,1.475; 7 0.5,1.475; 8 0,1.475; 9 -0.5,1.475; 10 -1,1.475 | smd 0.7 x 0.28: 11 -1.5,0.25; 12 -1.5,-0.25; 13 1.5,0.25; 14 1.5,-0.25 | smd 2.4 x 1.65: 15 0,0

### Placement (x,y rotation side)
BLDR-EN  54.93,11.43 0 top
C1  25.72,7.62 270 bottom
C2  50.48,22.23 270 bottom
C3  70.8,39.05 0 bottom
C4  59.69,34.29 90 bottom
C5  57.78,41.27 270 bottom
C8  13.97,22.86 270 bottom
C9  6.03,33.66 0 bottom
C10  6.35,36.83 90 bottom
C11  16.83,36.2 180 top
C12  13.34,26.99 90 bottom
C13  16.83,32.7 0 bottom
C14  14.61,18.73 180 bottom
C17  58.1,43.81 180 top
C18  60.33,41.27 90 bottom
C19  51.75,41.27 270 top
C20  54.93,43.81 180 top
C21  55.24,41.27 90 bottom
C22  52.7,31.75 0 bottom
C23  70.8,37.47 0 bottom
C24  60.96,17.14 90 bottom
C25  65.72,39.05 0 bottom
C26  52.7,30.16 0 bottom
C27  54.29,48.58 270 bottom
C28  55.88,48.58 270 bottom
C29  43.5,24.77 180 bottom
C30  43.5,23.18 180 bottom
C31  36.51,54.61 0 bottom
C32  36.51,53.02 0 bottom
C33  33.97,46.67 90 bottom
C34  32.38,46.67 90 bottom
C35  40.01,42.86 180 bottom
C36  40.01,44.45 180 bottom
C37  45.72,49.85 270 bottom
C38  44.13,49.85 270 bottom
C39  41.59,41.27 180 bottom
C40  44.77,45.72 270 bottom
C41  7.62,23.18 90 bottom
C42  9.21,23.18 90 bottom
DN1  8.26,30.34 90 top
DN2  7.94,18.73 90 top
IC1  39.05,48.26 180 top
IC2  55.56,28.57 90 top
IC3  56.52,49.53 0 top
J1  4.45,30 270 top
JP1  11.11,43.18 45 top
JP2  18.41,12.38 0 top
JP3  55.24,3.49 0 top
JP9  16.83,48.26 135 top
L1  18.73,22.54 0 top
LED1  28.26,55.88 180 top
LED2  25,30 180 top
Q3  50.48,22.23 270 top
Q4  26.67,7.62 270 top
Q5  14.61,18.73 0 top
Q6  60.96,17.14 90 top
Q7  65.72,39.05 180 top
R2  3.17,35.88 90 top
R3  57.15,33.97 180 top
R4  50.48,52.7 90 top
R5  8.89,36.83 270 bottom
R6  50.48,49.53 90 top
R7  50.48,46.35 90 top
R8  16.83,34.29 0 top
R9  61.59,46.35 270 top
R10  33.02,54.93 270 bottom
R11  13.65,34.29 0 top
R12  12.7,26.67 270 top
R13  61.91,49.53 270 top
R14  61.59,52.7 270 top
R15  49.21,18.73 180 top
R16  50.16,11.75 0 top
R17  13.02,29.53 270 top
R18  47.94,49.53 90 top
R19  14.61,17.46 0 bottom
R20  20,34.92 180 top
R21  21.59,31.75 90 top
R22  47.94,44.77 0 top
R23  45.4,42.23 0 top
R24  56.52,55.24 0 top
R25  55.24,41.27 270 top
R26  24.45,32.7 180 top
R27  28.57,30.16 270 top
R28  27.94,32.7 180 top
R29  53.66,41.27 270 top
R30  60.33,41.27 270 top
R31  57.78,41.27 270 top
R32  61.28,28.89 270 top
R33  54.29,23.5 180 top
R34  57.47,23.5 180 top
R35  48.58,54.93 90 top
R38  68.9,25.4 90 bottom
R39  64.45,13.97 0 top
R40  61.28,13.97 0 top
R41  70.8,37.47 0 top
RESET  54.93,18.1 180 top
S3  25,20 270 top
S4  25,40 90 top
ST  8.57,23.5 180 top
SV2  72.07,35.56 90 bottom
TP1  59.69,33.34 90 top
TP2  50.48,26.67 90 top
TP3  12.06,13.97 0 top
TP4  18.1,38.73 0 top
TP5  53.98,37.47 270 top
TP6  68.26,14.61 0 top
TP7  60.96,35.56 0 top
TP8  56.52,36.51 0 top
U1  7.62,36.83 270 top
U2  46.04,54.93 180 top
U3  43.81,9.53 180 top
U6  16.51,28.26 0 top

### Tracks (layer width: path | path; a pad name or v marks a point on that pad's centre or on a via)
3.3V1
  Top 0.305: U6.10 15.3,29.53 14.92,29.53 14.02,28.63 R17.2 13.02,27.57 R12.1
435
  Top 0.406: LED2.3 28.37,29.15 R27.2
+3V3  (via drill 0.6 pad 0.12)
  Top 0.305: U6.2 16.01,24.9 15.88,24.77
  Top 0.406: ST.8 7.37,22.53 C41.1
  Top 0.762: IC3.4 53.02,49.53 v52.07,48.58 | v48.26,56.83 48.58,56.52 R35.2 | SV2.VCC 72.07,37.09 C23.1 | IC2.8 v53.66,33.02 53.66,33.97 50.48,37.15 50.48,43.18 v52.07,44.77 | v42.23,26.35 42.55,26.02 U3.12 43.83,26.04 45.09,26.04 45.72,25.4 45.72,20 46.99,18.73 R15.2 | IC1.9 42.95,50.66 v42.86,50.75 | v37.47,56.52 37.47,54.07 IC1.19 | IC1.31 34.78,45.86 v34.92,45.72 | IC1.39 39.05,44.77 v40.01,45.72 | LED2.1 23.45,28.3 v23.81,27.94 | 15.88,24.77 13.39,24.77 v13.36,24.79 13.07,25.08 12.7,25.08 | 12.7,25.08 12.7,20.64 v12.06,20 TP3.TP 15.56,13.97 JP2.2 | C41.1 v7.62,21.27 | R12.2 12.7,25.08
  Bottom 0.508: C27.1 54.1,49.48 IC3.4
  Bottom 0.762: v52.07,48.58 49.85,48.58 47.62,50.8 45.77,50.8 C37.1 C38.1 v42.86,50.75 40.01,50.75 | 40.01,50.75 39.69,50.75 C32.1 C31.1 37.41,56.46 v37.47,56.52 41.27,56.52 41.59,56.83 43.18,56.83 43.5,56.52 47.94,56.52 v48.26,56.83 | v52.07,48.58 52.97,49.48 C27.1 C28.1 | C3.1 C23.1 71.7,35.93 | 71.7,35.93 SV2.VCC | 71.7,35.93 71.7,34.87 70.8,33.97 63.5,33.97 62.87,33.34 62.87,28.57 59.37,25.08 56.2,25.08 53.66,27.62 | 53.66,27.62 53.66,30.11 C26.1 | C26.1 C22.1 | v53.66,33.02 53.66,30.21 C26.1 | v52.07,44.77 v52.07,48.58 | 53.66,27.62 52.7,26.67 42.86,26.67 | 42.86,26.67 42.55,26.67 v42.23,26.35 | v42.23,26.35 42.23,25.14 C29.1 C30.1 | v42.23,26.35 42.55,26.35 42.86,26.67 | 40.01,50.75 37.47,48.21 37.47,46.41 | 40.01,45.67 v40.01,45.72 39.1,44.82 C36.1 | C35.1 C36.1 | 37.47,46.41 37.47,46.35 36.83,45.72 v34.92,45.72 34.02,45.72 C33.1 C34.1 32.33,45.72 32.38,45.72 32.07,45.4 32.07,34.29 25.72,27.94 v23.81,27.94 22.54,26.67 17.28,26.67 16.01,25.4 16.01,25.22 15.56,24.77 14.29,24.77 13.84,24.32 | C8.1 13.97,24.18 13.84,24.32 | 13.84,24.32 v13.36,24.79 | v7.62,21.27 C41.1 7.49,22.41 9.07,22.41 C42.1 9.79,22.28 v12.06,20 | 37.47,46.41 37.73,46.41 39.21,44.93 39.21,44.56 C36.1
ADC1
  Top 0.406: R23.1 43.28,42.23 IC1.44
ADC2
  Top 0.406: R24.1 55.62,51.8 55.24,51.44 52.39,51.44 52.07,51.12 52.07,49.85 51.75,49.53 49.85,49.53 49.21,48.9 49.21,46.67 47.94,45.4 47.94,44.13 47.62,43.81 45.3,43.81 IC1.1
ADC3
  Top 0.305: 46.75,45.06 R22.1
  Top 0.406: IC1.2 46.75,45.06
ADC4
  Top 0.406: R18.1 47.94,46.67 47.13,45.86 IC1.3
B  (via drill 0.6 pad 0.12)
  Top 0.406: IC1.20 36.65,55.74 35.56,56.83 32.07,56.83 v28.57,53.34 | v25.4,33.97 25.4,32.76 R26.1
  Bottom 0.406: v28.57,53.34 27.3,52.07 27.3,34.29 26.99,33.97 v25.4,33.97
B2
  Top 0.406: LED2.2 23.45,32.6 R26.2
BLDR-EN  (via drill 0.6 pad 0.12)
  Top 0.406: R16.1 48.9,11.75 45.09,7.94 42.55,7.94 35.24,15.24 v35.24,25.72 | v35.24,31.75 35.24,34.61 29.53,40.32 29.53,47.31 30.48,48.26 IC1.28
  Bottom 0.406: v35.24,25.72 v35.24,31.75
BT-EN  (via drill 0.6 pad 0.12)
  Top 0.406: IC1.13 42.23,54.06 42.23,52.7 38.1,48.58 38.1,44.77 v37.78,44.45
  Top 0.762: Q4.1 25.57,9.38 v25.72,9.53
  Bottom 0.406: v25.72,9.53 25.72,10.48 40.01,24.77 40.01,33.34 37.78,35.56 v37.78,44.45
  Bottom 0.762: v25.72,9.53 C1.1
BT-KEY  (via drill 0.6, 0.6 pad 0.12)
  Top 0.406: IC1.14 41.45,52.88 37.15,48.58 37.15,45.09 v36.51,44.45 | 30.75,21.59 U3.26 32.32,21.52 v32.7,21.91
  Bottom 0.406: v36.51,44.45 36.51,35.56 39.05,33.02 39.05,25.08 35.88,21.91 v32.7,21.91
BT-STAT  (via drill 0.6 pad 0.12)
  Top 0.406: U3.24 32.46,24.52 v32.7,24.77 | IC1.15 40.65,53.03 36.2,48.58 36.2,45.4 v35.24,44.45
  Bottom 0.406: v32.7,24.77 37.78,24.77 38.1,25.08 38.1,32.7 35.24,35.56 v35.24,44.45
C-STAT  (via drill 0.6 pad 0.12)
  Top 0.406: v6.35,39.05 6.32,39.02 U1.1 3.49,37.78 3.17,37.47 R2.2 | IC1.11 43.81,53.3 43.81,57.47 v44.13,57.78
  Bottom 0.406: v6.35,39.05 6.35,39.69 21.59,54.93 22.54,54.93 26.35,58.74 43.18,58.74 v44.13,57.78
D+  (via drill 0.6 pad 0.12)
  Top 0.406: v26.35,46.04 29.38,49.06 IC1.27 | 7.3,29.84 7.15,30 J1.3 | 7.3,29.84 DN1.1 | 7.3,29.84 7.62,30.16 10.48,30.16 v11.11,30.8
  Bottom 0.406: v11.11,30.8 v26.35,46.04
D-  (via drill 0.6 pad 0.12)
  Top 0.406: IC1.26 28.91,49.86 v26.35,47.31 | 7.3,30.9 DN1.6 | v11.11,32.07 9.84,30.8 7.4,30.8 7.3,30.9 | 7.3,30.9 7.05,30.65 J1.2
  Bottom 0.406: v26.35,47.31 v11.11,32.07
DATA-DHT
  Top 0.406: IC1.12 43.05,58.29 43.5,58.74 65.41,58.74 69.9,54.24 R41.1 69.53,37.09 SV2.SIG
DEBUG-RX
  Top 0.406: JP9.2 20.95,52.39 20.95,53.02 27.3,59.37 37.78,59.37 39.85,57.3 IC1.16
DEBUG-TX
  Top 0.406: JP9.1 18.83,46.67 19.05,46.67 22.23,49.85 22.23,53.02 27.62,58.42 37.47,58.42 39.05,56.83 IC1.17
G  (via drill 0.6 pad 0.12)
  Top 0.406: IC1.21 35.85,55.59 35.56,55.88 32.38,55.88 v29.84,53.34 | R28.1 28.84,33.92 v28.57,34.29
  Bottom 0.406: v28.57,34.29 28.57,52.07 v29.84,53.34
G2
  Top 0.406: LED2.4 26.72,30.85 26.99,31.11 26.99,32.65 R28.2
GND  (via drill 0.6 pad 0.12)
  Top 0.406: ST.4 10.48,24.46 v10.48,25.4 | v43.18,46.04 42.55,46.04 42.23,45.72 42.23,42.48 IC1.43
  Top 0.762: U1.2 v5.08,36.83 | Q3.2 47.94,21.27 v47.62,21.59
  Bottom 0.406: C40.2 44.4,44.82 v43.18,46.04
  Bottom 0.762: C2.2 47.89,21.32 v47.62,21.59
  other vias: 6.35,25.4 21.59,38.42 65.09,41.59 61.91,39.05 52.39,38.42 49.21,40.01 39.37,37.15 41.91,35.56 45.4,36.2 15.88,42.55 13.97,15.24
  pour Top: 0,40.01 0,20 20,0 74.93,0 74.93,60.01 20,60.01
  pour Bottom: 0,40.01 0,20 20,0 74.93,0 74.93,60.01 20,60.01
GND1
  Top 0.305: U6.9 16.01,30.34 15.88,30.48 13.07,30.48 R17.1
  Top 0.762: R11.1 12.75,30.69 R17.1
HY-EN  (via drill 0.6 pad 0.12)
  Top 0.406: v49.21,25.4 48.9,25.72 v48.9,28.89 | IC1.5 43.33,47.46 v43.18,47.31
  Top 0.762: v63.5,16.19 Q6.1
  Bottom 0.406: C24.1 59.64,16.25 50.8,25.08 49.53,25.08 v49.21,25.4 | v48.9,28.89 48.9,36.51 45.4,40.01 45.4,42.55 42.23,45.72 42.23,46.35 v43.18,47.31
  Bottom 0.762: C24.1 63.45,16.25 v63.5,16.19
LED  (via drill 0.6 pad 0.12)
  Top 0.406: IC1.23 33.25,52.79 v33.02,53.02
  Bottom 0.406: v33.02,53.02 R10.2
LIGHT-BUTTON  (via drill 0.6 pad 0.12)
  Top 0.406: IC1.24 27.65,51.46 v22.86,46.67 | ST.5 7.61,24.46 7.62,24.45 7.94,24.77 7.94,26.67 v7.62,26.99
  Bottom 0.406: v22.86,46.67 7.62,31.43 v7.62,26.99
LIGHT/WAKEUP-BUTTON1  (via drill 0.6 pad 0.12)
  Top 0.406: S4.T4 S4.T3 26.78,36.83 26.35,36.83 v25.08,35.56 | DN2.3 9.22,19.38 9.53,19.68 9.53,21.27 8.89,21.91 8.89,23.18 9.53,23.81 10.39,23.81 ST.3 9.51,23.82 9.21,24.13 9.21,26.04 v10.79,27.62
  Bottom 0.406: v10.79,27.62 13.34,30.16 17.46,30.16 22.54,35.24 24.77,35.24 v25.08,35.56
N$1
  Top 0.305: 50.75,52.07 R4.1
  Top 0.406: R6.2 R4.1 | IC3.2 50.75,52.07
N$2
  Top 0.305: 50.75,46.99 R7.2
  Top 0.406: IC3.6 50.75,46.99 | R7.2 R6.1
N$4
  Top 0.762: Q4.3 32.07,7.62 33.97,8.89 33.97,26.67 | 33.97,26.67 33.02,27.62 | 33.02,27.62 30.91,27.62 U3.22 | U3.21 32.06,27.62 33.02,27.62 | 33.97,26.67 34.92,27.62 43.72,27.62 U3.13
N$5
  Top 0.406: R16.2 51.06,10.34 BLDR-EN.T3 BLDR-EN.T4
N$6
  Bottom 0.406: R10.1 29.58,55.83 LED1.A
N$7
  Top 0.305: 61.33,46.99 R9.1 61.91,47.57 R13.2
  Top 0.406: IC3.9 61.33,46.99
N$8
  Top 0.305: U6.3 16.51,25.08 17.78,23.81 17.78,22.67 L1.P$1
N$9  (via drill 0.6 pad 0.12)
  Top 0.305: U6.1 15.51,26.62 v14.92,26.04
  Bottom 0.305: v14.92,26.04 13.6,26.04 C12.1
N$10  (via drill 0.6 pad 0.12)
  Top 0.406: DN2.2 v9.84,18.73 | Q5.1 13.65,17.73 13.71,17.78
  Top 0.762: v13.34,19.68 13.34,18.15 13.71,17.78
  Bottom 0.762: v9.84,18.73 C14.1 | C14.1 13.71,19.32 v13.34,19.68 | R19.2 C14.1
N$11  (via drill 0.6 pad 0.12)
  Top 0.762: U1.5 8.92,38.7 v8.89,38.73
  Bottom 0.762: v8.89,38.73 R5.1
N$12
  Top 0.305: 61.33,52.07 R14.2 61.86,51.8 61.91,51.75 R13.1
  Top 0.406: IC3.13 61.33,52.07
N$14
  Top 0.305: 50.75,53.34 R4.2 50.11,53.6
  Top 0.406: IC3.1 50.75,53.34 | 50.11,53.6 47.94,51.44 R18.2
N$15
  Top 0.406: IC3.7 50.75,45.72 R7.1 49.8,44.77 R22.2
N$19  (via drill 0.6 pad 0.12)
  Top 0.305: 61.33,45.72 R9.2
  Top 0.406: 61.33,45.72 IC3.8 59.37,45.72 v60.64,44.45 | v48.9,42.23 R23.2
  Bottom 0.406: v60.64,44.45 60.64,43.81 60.33,43.5 50.16,43.5 v48.9,42.23
N$21
  Top 0.305: 61.33,53.34 R14.1
  Top 0.406: 61.33,53.34 IC3.14 58.98,53.68 R24.2
N$22  (via drill 0.6 pad 0.12)
  Top 0.406: IC3.10 57.78,48.26 57.47,47.94 57.47,45.09 57.78,44.77 58.05,44.77 C17.1 59,43.5 C18.2 61.54,42.17 v61.59,42.23
  Bottom 0.406: v61.59,42.23 60.38,42.23 C18.2
N$23
  Top 0.406: IC2.3 56.2,23.86 R34.2 R33.1
N$25
  Top 0.406: IC3.5 55.24,48.26 55.56,47.94 55.56,45.09 55.24,44.77 54.98,44.77 C20.2 54.03,42.55 R29.1 C19.1
N$26  (via drill 0.6 pad 0.12)
  Top 0.406: IC3.3 55.24,50.8 56.2,49.85 56.2,44.77 55.83,44.4 C20.1 55.83,42.76 R25.1 56.46,42.17 v56.52,42.23
  Bottom 0.406: v56.52,42.23 55.3,42.23 R25.1
N$27  (via drill 0.6 pad 0.12)
  Top 0.406: IC3.12 57.78,50.8 56.83,49.85 56.83,44.77 57.2,44.4 C17.2 57.2,42.76 R31.1 57.84,42.23 v59.05,42.23
  Bottom 0.406: R31.1 59,42.17 v59.05,42.23
N$28
  Top 0.762: JP3.2 60.24,6.59 66.99,13.34 | 66.99,13.34 TP6.TP 71.44,14.61 74.3,17.46 74.3,21.27 73.98,21.59 R38.8 | R39.2 66.36,13.97 66.99,13.34
N$29
  Top 0.762: R40.1 59.86,14.49 Q6.3 60.01,17.29 60.01,20.64 60.96,21.59 R38.1
N$30
  Top 0.762: Q7.3 65.72,36.83 SV2.GND
N$33
  Top 0.305: 60.33,35.24 60.64,35.24 TP7.TP
  Top 0.406: 61.91,33.02 73.98,33.02 74.3,32.7 74.3,24.45 73.98,24.13 R38.7 | R32.1 61.28,32.38 61.91,33.02 | R29.2 53.66,40.96 53.98,41.27 59.42,41.27 R30.2 60.33,35.24 61.91,33.66 61.91,33.02
N$34
  Top 0.406: R25.2 55.24,38.73 TP5.TP 53.98,35.24 54.93,34.29 IC2.7 54.93,29.84 56.78,27.99 R32.2
N$35
  Top 0.406: R31.2 57.78,39.69 56.25,38.15 56.25,36.51 | R38.2 62.87,24.13 62.55,24.45 62.55,28.57 62.23,28.89 57.47,28.89 56.2,30.16 IC2.6 56.2,33.92 R3.2 56.25,35.88 56.25,36.51 | TP8.TP 56.25,36.51
ON-BUTTON  (via drill 0.6 pad 0.12)
  Top 0.406: IC1.25 28.12,50.66 v24.13,46.67 | ST.7 7.92,23.16 8.57,23.81 8.57,26.67 v8.89,26.99
  Bottom 0.406: v24.13,46.67 8.89,31.43 v8.89,26.99
PAD@4  (via drill 0.6 pad 0.12)
  Top 0.305: U6.12 U6.11 16.26,28.51 U6.15 | U6.13 U6.14 | U6.15 16.83,28.26 | 16.83,28.26 17.14,28.57 17.21,28.51 U6.13 | 16.83,28.26 16.83,27.94 | U6.15 17.01,27.76 U6.4 17.01,25.85 v17.46,25.4 | U6.13 18.01,29.12 v18.41,29.53
  Top 0.762: v21.59,29.53 R21.1 | v17.46,19.68 17.32,19.83 Q5.3
  Bottom 0.762: v18.41,29.53 v21.59,29.53 | v17.46,25.4 v17.46,19.68
PDI_DATA  (via drill 0.6 pad 0.12)
  Top 0.406: IC1.34 35.05,41.09 v34.29,40.32
  Bottom 0.406: v34.29,40.32 34.29,33.02 17.14,15.88 17.14,12.38 JP2.1
POWER-EN  (via drill 0.6 pad 0.12)
  Top 0.406: IC1.29 31.27,47.46 v30.8,46.99 | v30.8,36.2 33.02,33.97 v33.02,33.34 | v6.03,17.46 6.65,18.08 DN2.5
  Bottom 0.406: v30.8,46.99 v30.8,36.2 | v33.02,33.34 15.88,16.19 6.67,16.19 6.03,16.83 v6.03,17.46
R  (via drill 0.6 pad 0.12)
  Top 0.406: IC1.22 35.05,54.8 34.92,54.93 32.7,54.93 v31.11,53.34 | R27.1 29.16,31.06 29.84,31.75 v29.84,33.97
  Bottom 0.406: v31.11,53.34 29.84,52.07 v29.84,33.97
RST/PDI_CLK
  Top 0.406: RESET.T3 RESET.T4 50.61,18.73 R15.1 50.11,19.1 | RESET.T3 58.37,19.95 58.42,20 58.08,20 RESET.T3 | 50.11,19.1 49.21,20 47.31,20 46.67,20.64 46.67,31.11 44.13,33.66 40.01,33.66 35.88,37.78 35.88,41.91 35.85,41.94 IC1.35 | 50.11,19.1 50.16,19.05 50.16,10.48 44.77,5.08 23.81,5.08 20.95,7.94 JP2.5
RX-TX(BT)  (via drill 0.6 pad 0.12)
  Top 0.406: U3.1 42.55,9.53 36.2,15.88 v36.2,26.35 | v36.2,32.7 36.2,34.92 31.75,39.37 31.75,44.77 32.07,45.09 32.09,45.06 IC1.32
  Bottom 0.406: v36.2,26.35 v36.2,32.7
SEN1-EN  (via drill 0.6 pad 0.12)
  Top 0.406: v66.67,41.59 | v66.67,41.59 66.67,43.18 65.72,44.13 63.82,44.13 62.55,42.86 v62.55,41.27 | IC1.7 43.02,49.06 42.86,49.21 41.27,49.21 v40.96,48.9
  Top 0.762: Q7.1 v66.67,41.59
  Bottom 0.406: v62.55,41.27 48.58,41.27 47.94,41.91 47.94,42.86 48.9,43.81 48.9,47.62 46.67,49.85 41.91,49.85 v40.96,48.9
  Bottom 0.762: v66.67,41.59 66.67,39.1 C25.1
SEN2-EN  (via drill 0.6 pad 0.12)
  Top 0.406: v48.26,23.18 47.62,23.81 v47.62,29.84 | v42.23,48.26 IC1.6
  Top 0.762: Q3.1 v48.26,23.18
  Bottom 0.406: v47.62,29.84 47.62,36.2 44.45,39.37 44.45,42.23 42.23,44.45 42.23,44.77 41.27,45.72 41.27,47.31 v42.23,48.26
  Bottom 0.762: v48.26,23.18 50.43,23.18 C2.1
SEN-GND  (via drill 0.6 pad 0.12)
  Top 0.508: v50.16,54.93 47.62,54.93 47.31,55.24 47.31,55.69 U2.2
  Top 0.762: IC3.11 v60.64,49.53 | Q3.3 57.78,22.23 58.42,22.86 58.42,23.44 R34.1 58.37,25.21 IC2.4 57.86,26.11 v58.74,26.99 | R3.1 58.1,34.02 58.1,36.2 v59.05,37.15
  Bottom 0.762: v50.16,54.93 59.05,54.93 61.28,52.7 61.28,50.16 v60.64,49.53 63.82,46.35 63.82,38.1 61.59,35.88 | v58.74,26.99 61.59,29.84 61.59,35.88 | 61.59,35.88 60.33,37.15 v59.05,37.15
TX-RX(BT)  (via drill 0.6 pad 0.12)
  Top 0.406: U3.2 42.31,11.03 37.15,16.19 v37.15,25.72 | v37.15,31.75 37.15,35.24 33.34,39.05 33.34,44.17 IC1.33
  Bottom 0.406: v37.15,25.72 v37.15,31.75
USB-STAT  (via drill 0.6 pad 0.12)
  Top 0.406: IC1.10 44.11,51.46 43.5,52.07 v42.86,52.07 | v40.64,57.78 40.64,56.83 v41.91,55.56 | ST.2 11.42,23.16 11.75,23.5 11.75,24.77 11.43,25.08 11.43,26.04 v11.11,26.35
  Bottom 0.406: v42.86,52.07 41.91,53.02 v41.91,55.56 | v40.64,57.78 40.32,58.1 26.99,58.1 20,51.12 20,49.53 12.06,41.59 12.06,37.15 6.35,31.43 6.35,26.99 7.3,26.04 9.53,26.04 9.84,26.35 v11.11,26.35
UVLO1  (via drill 0.6 pad 0.12)
  Top 0.305: U6.7 17.01,31.3 v17.14,31.43 | R8.1 15.93,34.02 14.92,33.02 v14.92,31.75
  Top 0.406: R11.2 R8.1 C11.2
  Bottom 0.305: v17.14,31.43 16.51,31.75 v14.92,31.75
V-B  (via drill 0.6 pad 0.12)
  Top 0.305: 18.73,32.38 16.83,32.38 16.19,31.75 16.19,31.11 16.51,30.8 U6.8 | U6.6 17.51,30.21 18.73,31.43 | U6.5 17.51,26.62 18.41,25.72 19.37,25.72
  Top 0.762: JP1.1 13.02,39.69 | 13.02,39.69 10.16,36.83 7.94,36.83 7.62,36.51 7.62,36.2 7.3,35.88 U1.3 5.72,35.88 v5.08,35.24 | 13.02,39.69 13.33,39.69 14.92,38.1 17.46,38.1 | TP4.TP 17.46,38.1 | 17.46,38.1 17.46,37.78 17.78,37.47 17.78,36.25 C11.1 18.41,36.2 19.05,35.56 | 19.05,35.56 19.05,34.98 R20.2 19.05,34.92 18.41,34.29 | 18.41,34.29 R8.2 | 19.05,35.56 20.32,36.83 23.08,36.83 S4.T1 S4.T2 | 18.41,34.29 18.73,33.97 v18.73,33.02 18.73,32.38 18.73,31.43 19.68,30.48 19.68,26.04 19.37,25.72 19.68,25.4 19.68,22.67 L1.P$2 20,22.54 22.23,24.77 25.18,24.77 S3.T1 S3.T2
  Bottom 0.762: 18.1,33.02 18.05,33.02 C13.1 17.78,32.7 18.1,33.02 | 18.1,33.02 v18.73,33.02 | v5.08,35.24 5.71,35.88 6.3,35.88 C10.1
V-BATT  (via drill 0.6 pad 0.12)
  Top 0.406: IC1.41 40.65,40.31 v43.18,37.78 | v43.18,32.07 43.18,31.75 42.23,30.8 31.11,30.8 30.48,30.16 30.48,29.53 27.62,26.67 22.54,26.67 20.64,28.57 20.64,31.7 R21.2 21.59,34.24 R20.1
  Bottom 0.406: v43.18,37.78 v43.18,32.07
V-BATT-H  (via drill 0.6 pad 0.12)
  Top 0.406: R40.2 62.18,13.28 v61.59,12.7 | IC1.42 41.45,40.78 v42.23,40.01
  Top 0.762: R40.2 R39.1
  Bottom 0.406: v61.59,12.7 43.81,12.7 40.96,15.56 40.96,38.73 v42.23,40.01
V-REF  (via drill 0.6 pad 0.12)
  Top 0.406: IC2.2 IC2.1 53.66,28.26 | 53.66,28.26 51.75,30.16 49.53,30.16 39.37,40.32 v39.37,40.64 39.85,41.12 IC1.40 | 53.66,28.26 54.61,28.26 v54.93,28.57 | v59.05,30.8 59.05,31.11 58.74,31.43 | 57.86,31.43 IC2.5 57.47,31.11 57.78,31.43 57.86,31.43 | 57.86,31.43 58.74,31.43 | 58.74,31.43 v59.37,32.07
  Top 0.508: v59.37,32.07 59.37,33.02 TP1.TP
  Bottom 0.406: v54.93,28.57 56.83,28.57 v59.05,30.8 | C39.1 40.06,40.64 v39.37,40.64
  Bottom 0.508: C4.1 59.69,32.38 v59.37,32.07
V-REF-B  (via drill 0.6 pad 0.12)
  Top 0.406: IC1.4 46.34,46.66 v46.67,46.99 46.67,53.53 U2.1 48.54,53.99 R35.1 | R33.2 53.39,23.76 TP2.TP v50.48,29.21
  Bottom 0.406: C40.1 46.3,46.62 | 46.3,46.62 v46.67,46.99 | 46.3,46.62 46.41,46.62 46.67,46.35 46.67,40.32 50.48,36.51 v50.48,29.21
VUSB  (via drill 0.6, 0.6 pad 0.12)
  Top 0.508: 5.73,23.82 ST.6 | J1.1 5.58,31.3 6.03,31.75 v6.03,32.38
  Top 0.762: DN2.4 5.08,21.44 5.08,23.18 5.73,23.82 5.11,24.45 v5.08,24.45 | U1.4 8.52,35.48 8.49,35.48 v7.94,34.92 | v7.94,34.92 8.57,34.29 8.57,33.34 7.94,32.7 | v7.94,34.92 6.93,33.92 4.23,33.92 R2.1 | 7.94,32.7 6.35,32.7 v6.03,32.38 | 7.94,32.7 8.26,32.07 DN1.5
  Bottom 0.762: v7.94,34.92 7.94,34.66 C9.1 | v6.03,32.38 5.08,31.43 v5.08,24.45
WAKEUP-BUTTON1
  Top 0.406: S3.T4 S3.T3 23.15,16.48 22.86,16.19 18.73,16.19 17.14,14.61 17.14,12.7 16.83,12.38 11.43,12.38 10.48,13.34 10.48,17.78 | DN2.1 8.9,18.08 9.21,17.78 10.48,17.78 | 10.48,17.78 10.79,18.1 10.79,20.95 11.43,21.59 11.43,22.23 11.11,22.54 10.41,22.54 ST.1

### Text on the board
tNames: GND | RX | SNUFFELNEUS V1.0 | TX | DESIGNED BY: | P&P | GND | V+ | 3.3V | GND | DATA | R/CLK | GND | 12V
